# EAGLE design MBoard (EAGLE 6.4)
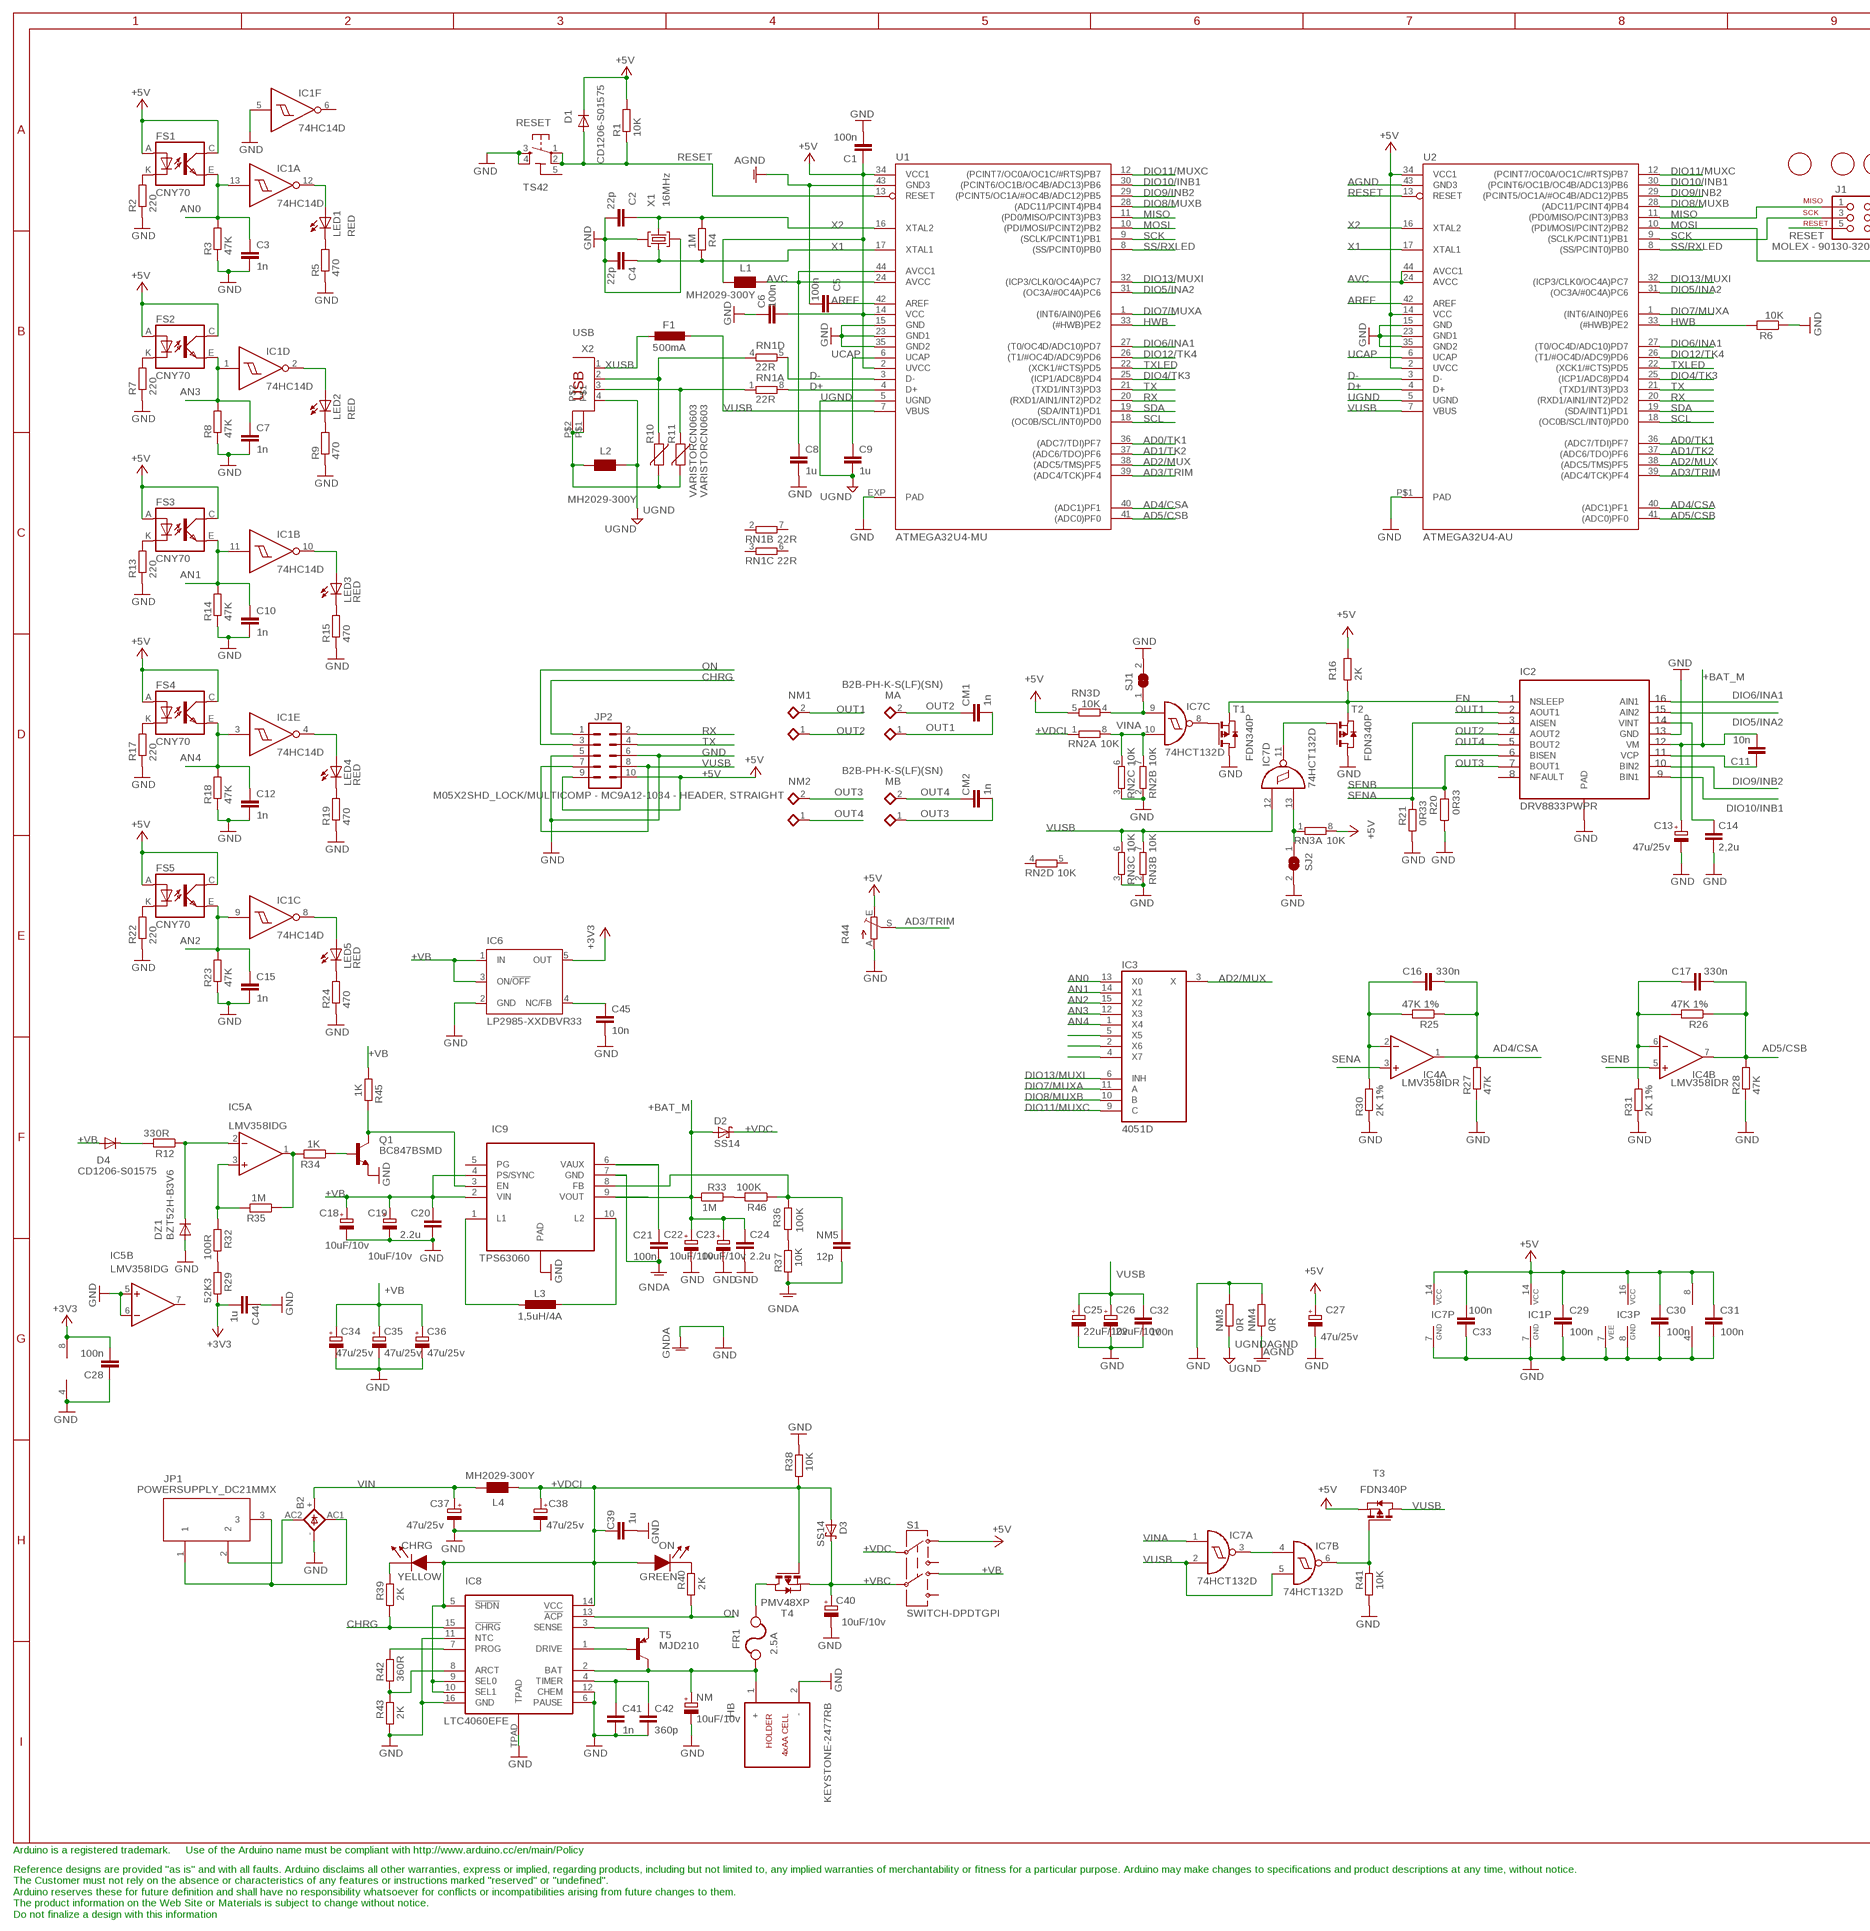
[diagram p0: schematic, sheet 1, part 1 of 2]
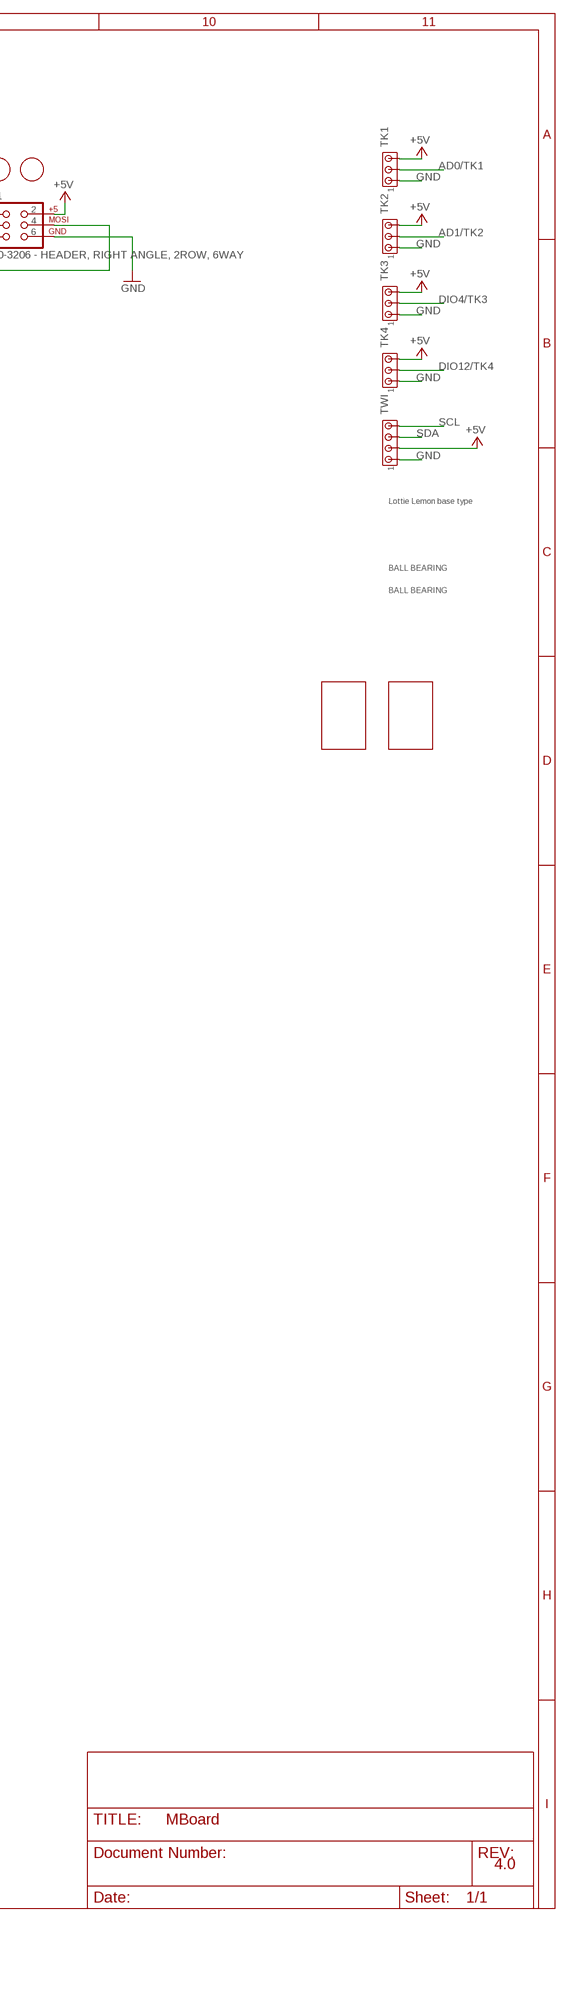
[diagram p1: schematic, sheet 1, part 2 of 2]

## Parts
B2  KBL  [KBL]
BB1  LOTTIE_LEMON_BALL_BEARING  [BALL_BEARING_LOTTIE_LEMON]
BB2  LOTTIE_LEMON_BALL_BEARING  [BALL_BEARING_LOTTIE_LEMON]
C1  100n  C-EUC0603  [C0603-ROUND]
C2  22p  C-EUC0603  [C0603-ROUND]
C3  1n  C-EUC0603  [C0603-ROUND]
C4  22p  C-EUC0603  [C0603-ROUND]
C5  100n  C-EUC0603  [C0603-ROUND]
C6  100n  C-EUC0603  [C0603-ROUND]
C7  1n  C-EUC0603  [C0603-ROUND]
C8  1u  C-EUC0603  [C0603-ROUND]
C9  1u  C-EUC0603  [C0603-ROUND]
C10  1n  C-EUC0603  [C0603-ROUND]
C11  10n  C-EUC0603  [C0603-ROUND]
C12  1n  C-EUC0603  [C0603-ROUND]
C13  47u/25v  CPOL-EUD  [PANASONIC_D]
C14  2,2u  C-EUC0805K  [C0805K]
C15  1n  C-EUC0603  [C0603-ROUND]
C16  330n  C-EUC0603  [C0603-ROUND]
C17  330n  C-EUC0603  [C0603-ROUND]
C18  10uF/10v  CPOL-EUSMCB  [SMC_B]
C19  10uF/10v  CPOL-EUSMCB  [SMC_B]
C20  2.2u  C-EUC0805K  [C0805K]
C21  100n  C-EUC0603  [C0603-ROUND]
C22  10uF/10v  CPOL-EUSMCB  [SMC_B]
C23  10uF/10v  CPOL-EUSMCB  [SMC_B]
C24  2.2u  C-EUC0805K  [C0805K]
C25  22uF/10v  CPOL-EUSMCB  [SMC_B]
C26  22uF/10v  CPOL-EUSMCB  [SMC_B]
C27  47u/25v  CPOL-EUD  [PANASONIC_D]
C28  100n  C-EUC0603  [C0603-ROUND]
C29  100n  C-EUC0603  [C0603-ROUND]
C30  100n  C-EUC0603  [C0603-ROUND]
C31  100n  C-EUC0603  [C0603-ROUND]
C32  100n  C-EUC0603  [C0603-ROUND]
C33  100n  C-EUC0603  [C0603-ROUND]
C34  47u/25v  CPOL-EUD  [PANASONIC_D]
C35  47u/25v  CPOL-EUD  [PANASONIC_D]
C36  47u/25v  CPOL-EUD  [PANASONIC_D]
C37  47u/25v  CPOL-EUD  [PANASONIC_D]
C38  47u/25v  CPOL-EUD  [PANASONIC_D]
C39  1u  C-EUC0603  [C0603-ROUND]
C40  10uF/10v  CPOL-EUSMCB  [SMC_B]
C41  1n  C-EUC0603  [C0603-ROUND]
C42  360p  C-EUC0603  [C0603-ROUND]
C44  1u  C-EUC0603  [C0603-ROUND]
C45  10n  C-EU0603-RND  [C0603-ROUND]
CHRG  YELLOW  MYSMD_LED0805  [SMD_LED0805]
CM1  1n  C-EUC0603  [C0603-ROUND]
CM2  1n  C-EUC0603  [C0603-ROUND]
D1  CD1206-S01575  DIODE-MINIMELF  [MINIMELF]
D2  SS14  SCHOTTKY-DIODESMD  [SMB@1]
D3  SS14  SCHOTTKY-DIODESMD  [SMB@1]
D4  CD1206-S01575  DIODE-MINIMELF  [MINIMELF]
DZ1  BZT52H-B3V6  DIODE-SOD123  [SOD123]
F1  500mA  L-EUL1812  [L1812]
FM1  FIDUCIALMOUNT  [FIDUCIA-MOUNT]
FM2  FIDUCIALMOUNT  [FIDUCIA-MOUNT]
FM3  FIDUCIALMOUNT  [FIDUCIA-MOUNT]
FR1  2.5A  PTC_RESETTABLE_FUSES  [MF-MSMF-S2]
FS1  CNY70  [4]
FS2  CNY70  [4]
FS3  CNY70  [4]
FS4  CNY70  [4]
FS5  CNY70  [4]
HB  KEYSTONE-2477RB  4XAA-BATTERY_HOLDER  [4XAA_BATTERY-HOLDER]
IC1  74HC14D  [SO14]
IC2  DRV8833PWPR  DRV8833  [R-PDSO-G16]
IC3  4051D  [SO16]
IC4  LMV358IDR  LMV358MX  [SO08@1]
IC5  LMV358IDG  LM358D  [SO08]
IC6  LP2985-XXDBVR33  [SOT23-DBV]
IC7  74HCT132D  [SO14]
IC8  LTC4060EFE  LTC4060  [TSSOP16]
IC9  TPS63060  [R-PVSON-10N]
J1  MOLEX - 90130-3206 - HEADER, RIGHT ANGLE, 2ROW, 6WAY  AVR_SPI_PRG_6PTH  [2X3]
JP1  POWERSUPPLY_DC21MMX  [POWERSUPPLY_DC-21MM]
JP2  M05X2SHD_LOCK/MULTICOMP - MC9A12-1034 - HEADER, STRAIGHT  M05X2SHD_LOCK  [2X5-SHROUDED_LOCK]
L1  MH2029-300Y  WE-CBF_0805  [0805]
L2  MH2029-300Y  WE-CBF_0805  [0805]
L3  1,5uH/4A  L-EUWE-TPC  [POWER-CHOKE_WE-TPC]
L4  MH2029-300Y  WE-CBF_0805  [0805]
LED1  RED  LEDCHIP-LED0805  [CHIP-LED0805]
LED2  RED  LEDCHIP-LED0805  [CHIP-LED0805]
LED3  RED  LEDCHIP-LED0805  [CHIP-LED0805]
LED4  RED  LEDCHIP-LED0805  [CHIP-LED0805]
LED5  RED  LEDCHIP-LED0805  [CHIP-LED0805]
LL1  LOTTIE_LEMON_DC_MOTOR_48X_L  [CARCASA_MOTOR_L_LOTTIE_LEMON]
MA  B2B-PH-K-S(LF)(SN)  B2B-PH-KL  [B2B-PH_KL]
MB  B2B-PH-K-S(LF)(SN)  B2B-PH-KL  [B2B-PH_KL]
NM  10uF/10v  CPOL-EUSMCB  [SMC_B]
NM1  B2B-PH-K-S(LF)(SN)  B2B-PH-KL  [B2B-PH_KL]
NM2  B2B-PH-K-S(LF)(SN)  B2B-PH-KL  [B2B-PH_KL]
NM3  0R  R-EU_R0805  [R0805]
NM4  0R  R-EU_R0805  [R0805]
NM5  12p  C-EUC0603  [C0603-ROUND]
ON  GREEN  MYSMD_LED0805  [SMD_LED0805]
Q1  BC847BSMD  [SOT23]
R1  10K  R-EU_0603-RND  [R0603-ROUND]
R2  220  R-EU_R0603  [R0603-ROUND]
R3  47K  R-EU_R0603  [R0603-ROUND]
R4  1M  R-EU_0603-RND  [R0603-ROUND]
R5  470  R-EU_R0603  [R0603-ROUND]
R6  10K  R-EU_0603-RND  [R0603-ROUND]
R7  220  R-EU_R0603  [R0603-ROUND]
R8  47K  R-EU_0603-RND  [R0603-ROUND]
R9  470  R-EU_0603-RND  [R0603-ROUND]
R10  VARISTORCN0603  [CT/CN0603]
R11  VARISTORCN0603  [CT/CN0603]
R12  330R  R-EU_0603-RND  [R0603-ROUND]
R13  220  R-EU_R0603  [R0603-ROUND]
R14  47K  R-EU_R0603  [R0603-ROUND]
R15  470  R-EU_R0603  [R0603-ROUND]
R16  2K  R-EU_0603-RND  [R0603-ROUND]
R17  220  R-EU_R0603  [R0603-ROUND]
R18  47K  R-EU_R0603  [R0603-ROUND]
R19  470  R-EU_R0603  [R0603-ROUND]
R20  0R33  R-EU_R1206  [R1206]
R21  0R33  R-EU_R1206  [R1206]
R22  220  R-EU_R0603  [R0603-ROUND]
R23  47K  R-EU_R0603  [R0603-ROUND]
R24  470  R-EU_R0603  [R0603-ROUND]
R25  47K 1%  R-EU_0603-RND  [R0603-ROUND]
R26  47K 1%  R-EU_0603-RND  [R0603-ROUND]
R27  47K  R-EU_0603-RND  [R0603-ROUND]
R28  47K  R-EU_0603-RND  [R0603-ROUND]
R29  52K3  R-EU_0603-RND  [R0603-ROUND]
R30  2K 1%  R-EU_0603-RND  [R0603-ROUND]
R31  2K 1%  R-EU_0603-RND  [R0603-ROUND]
R32  100R  R-EU_0603-RND  [R0603-ROUND]
R33  1M  R-EU_0603-RND  [R0603-ROUND]
R34  1K  R-EU_0603-RND  [R0603-ROUND]
R35  1M  R-EU_0603-RND  [R0603-ROUND]
R36  100K  R-EU_0603-RND  [R0603-ROUND]
R37  10K  R-EU_0603-RND  [R0603-ROUND]
R38  10K  R-EU_0603-RND  [R0603-ROUND]
R39  2K  R-EU_0603-RND  [R0603-ROUND]
R40  2K  R-EU_0603-RND  [R0603-ROUND]
R41  10K  R-EU_0603-RND  [R0603-ROUND]
R42  360R  R-EU_0603-RND  [R0603-ROUND]
R43  2K  R-EU_0603-RND  [R0603-ROUND]
R44  TRIM_EU-CA9V  [CA9V]
R45  1K  R-EU_0603-RND  [R0603-ROUND]
R46  100K  R-EU_0603-RND  [R0603-ROUND]
RESET  TS42  [TS42]
RN1  22R  4R-NCAY16  [CAY16]
RN2  10K  4R-NCAY16  [CAY16]
RN3  10K  4R-NCAY16  [CAY16]
RR1  LOTTIE_LEMON_DC_MOTOR_48X_R  [CARCASA_MOTOR_R_LOTTIE_LEMON]
S1  SWITCH-DPDTGPI  [GPI-152-3013]
SJ1  SJL  [SJL]
SJ2  SJL  [SJL]
T1  FDN340P  PMOSSOT23  [SOT-23]
T2  FDN340P  PMOSSOT23  [SOT-23]
T3  FDN340P  PMOSSOT23  [SOT-23]
T4  PMV48XP  PMOSSOT23  [SOT-23]
T5  MJD210  MJD32  [DPAK]
TK1  MTA03-100  [10X03MTA]
TK2  MTA03-100  [10X03MTA]
TK3  MTA03-100  [10X03MTA]
TK4  MTA03-100  [10X03MTA]
TWI  MTA04-100  [10X04MTA]
U1  ATMEGA32U4-MU  ATMEGA32U4-XUMU  [QFN44ML7X7]
U2  ATMEGA32U4-AU  ATMEGA32U4-XUAU  [TQFP44-PAD]
U$1  LOTTIE_LEMON_BASE_TYPE  [BASE_ROBOT_001]
U$2  LOTTIE_LEMON_PADS  [PADS_LOTTIE_LEMON]
W1  LOTTIE_LEMON_WHEEL  [WHEEL_LOTTIE_LEMON]
W2  LOTTIE_LEMON_WHEEL  [WHEEL_LOTTIE_LEMON]
X1  16MHz  CRYSTAL-3.2-2.5  [CRYSTAL-3.2-2.5]
X2  USB  PN61729  [PN61729]

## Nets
+3V3: C28.2 C44.1 IC5.8(P:V+) IC6.5(OUT) R29.2
+5V [+5v]: C1.1 C6.2 C27.+ C29.1 C30.1 C31.1 C33.2 D1.C FS1.A FS1.C(COL) FS2.A FS2.C(COL) FS3.A FS3.C(COL) FS4.A FS4.C(COL) FS5.A FS5.C(COL) IC1.14(P:VCC) IC3.16(VCC) IC4.8(P:V+) IC7.14(P:VCC) J1.2 JP2.9 JP2.10 L1.1 R1.2 R16.2 R44.E RN3.5 RN3.8 S1.10 T3.2(S) TK1.3 TK2.3 TK3.3 TK4.3 TWI.2 U1.2(UVCC) U1.14(VCC) U1.34(VCC1) U2.2(UVCC) U2.14(VCC) U2.34(VCC1)
+BAT_M [power]: C11.2 C13.+ C22.+ C23.+ C24.1 D2.A IC2.P$12(VM) IC9.9(VOUT) R33.1
+VB [power]: C18.+ C19.+ C20.1 C34.+ C35.+ C36.+ D4.A IC6.1(IN) IC6.3(ON/!OFF) IC9.2(VIN) IC9.4(PS/SYNC) R45.1 S1.11
+VBC [+5v]: C40.+ D3.C S1.C@2 T4.2(S)
+VDC [+5v]: D2.C S1.C@1
+VDCI [power]: C38.+ C39.2 CHRG.2(AN) D3.A IC8.5(!SHDN) IC8.9(SEL0) IC8.10(SEL1) IC8.14(VCC) L4.2 ON.2(AN) R38.1 RN2.1 T4.3(G)
AD0/TK1: TK1.2 U1.36((ADC7/TDI)PF7) U2.36((ADC7/TDI)PF7)
AD1/TK2: TK2.2 U1.37((ADC6/TDO)PF6) U2.37((ADC6/TDO)PF6)
AD2/MUX: IC3.3(X) U1.38((ADC5/TMS)PF5) U2.38((ADC5/TMS)PF5)
AD3/TRIM: R44.S U1.39((ADC4/TCK)PF4) U2.39((ADC4/TCK)PF4)
AD4/CSA: C16.2 IC4.1(A:OUT) R25.1 R27.2 U1.40((ADC1)PF1) U2.40((ADC1)PF1)
AD5/CSB: C17.2 IC4.7(B:OUT) R26.1 R28.2 U1.41((ADC0)PF0) U2.41((ADC0)PF0)
AGND: C5.2 NM4.1 U1.43(GND3) U2.43(GND3)
AN0: C3.1 FS1.E(EMI) IC1.13(A:I) IC3.13(X0) R3.2
AN1: C10.1 FS3.E(EMI) IC1.11(B:I) IC3.14(X1) R14.2
AN2: C15.1 FS5.E(EMI) IC1.9(C:I) IC3.15(X2) R23.2
AN3: C7.1 FS2.E(EMI) IC1.1(D:I) IC3.12(X3) R8.2
AN4: C12.1 FS4.E(EMI) IC1.3(E:I) IC3.1(X4) R18.2
AREF: C5.1 U1.42(AREF) U2.42(AREF)
AVC: C8.1 L1.2 U1.24(AVCC) U1.44(AVCC1) U2.24(AVCC) U2.44(AVCC1)
CHRG: IC8.15(!CHRG) JP2.1 R39.1
D+: RN1.8 U1.4(D+) U2.4(D+)
D-: RN1.5 U1.3(D-) U2.3(D-)
DIO4/TK3: TK3.2 U1.25((ICP1/ADC8)PD4) U2.25((ICP1/ADC8)PD4)
DIO5/INA2: IC2.P$15(AIN2) U1.31((OC3A/#0C4A)PC6) U2.31((OC3A/#0C4A)PC6)
DIO6/INA1: IC2.P$16(AIN1) U1.27((T0/OC4D/ADC10)PD7) U2.27((T0/OC4D/ADC10)PD7)
DIO7/MUXA: IC3.11(A) U1.1((INT6/AIN0)PE6) U2.1((INT6/AIN0)PE6)
DIO8/MUXB: IC3.10(B) U1.28((ADC11/PCINT4)PB4) U2.28((ADC11/PCINT4)PB4)
DIO9/INB2: IC2.P$10(BIN2) U1.29((PCINT5/OC1A/#OC4B/ADC12)PB5) U2.29((PCINT5/OC1A/#OC4B/ADC12)PB5)
DIO10/INB1: IC2.P$9(BIN1) U1.30((PCINT6/OC1B/OC4B/ADC13)PB6) U2.30((PCINT6/OC1B/OC4B/ADC13)PB6)
DIO11/MUXC: IC3.9(C) U1.12((PCINT7/OC0A/OC1C/#RTS)PB7) U2.12((PCINT7/OC0A/OC1C/#RTS)PB7)
DIO12/TK4: TK4.2 U1.26((T1/#OC4D/ADC9)PD6) U2.26((T1/#OC4D/ADC9)PD6)
DIO13/MUXI: IC3.6(INH) U1.32((ICP3/CLK0/OC4A)PC7) U2.32((ICP3/CLK0/OC4A)PC7)
EN [+5v]: IC2.P$1(NSLEEP) R16.1 T1.2(S) T2.2(S)
GND [gnd]: B2.- C1.2 C2.2 C3.2 C4.2 C6.1 C7.2 C8.2 C10.2 C12.2 C13.- C14.2 C15.2 C18.- C19.- C20.2 C22.- C23.- C24.2 C25.- C26.- C27.- C28.1 C29.2 C30.2 C31.2 C32.1 C33.1 C34.- C35.- C36.- C37.- C38.- C39.1 C40.- C41.2 C42.2 C44.2 C45.2 DZ1.A HB.2(-) IC1.5(F:I) IC1.7(P:GND) IC2.P$13(GND) IC2.P$17(PAD) IC3.7(VEE) IC3.8(GND) IC4.4(P:V-) IC5.4(P:V-) IC5.5(B:+IN) IC5.6(B:-IN) IC6.2(GND) IC7.7(P:GND) IC8.6(PAUSE) IC8.11(NTC) IC8.12(CHEM) IC8.16(GND) IC8.TPAD IC9.PAD J1.6 JP2.5 JP2.6 NM3.2 NM4.2 NM.- Q1.2(E) R2.1 R3.1 R5.1 R6.1 R7.1 R8.1 R9.1 R13.1 R14.1 R15.1 R17.1 R18.1 R19.1 R20.1 R21.1 R22.1 R23.1 R24.1 R27.1 R28.1 R30.1 R31.1 R38.2 R41.1 R43.1 R44.A RESET.3 RESET.4 RN2.2 RN2.3 RN3.2 RN3.3 SJ1.2 SJ2.2 T1.1(D) T2.1(D) TK1.1 TK2.1 TK3.1 TK4.1 TWI.1 U1.15(GND) U1.23(GND1) U1.35(GND2) U1.EXP(PAD) U2.15(GND) U2.23(GND1) U2.35(GND2) U2.P$1(PAD) X1.2(GND) X1.4(GND)
GNDA [gnd]: C21.2 IC9.7(GND) NM5.2 R37.1 ; supply symbol labelled GND
HWB: R6.2 U1.33((#HWB)PE2) U2.33((#HWB)PE2)
MISO: J1.1 U1.11((PD0/MISO/PCINT3)PB3) U2.11((PD0/MISO/PCINT3)PB3)
MOSI: J1.4 U1.10((PDI/MOSI/PCINT2)PB2) U2.10((PDI/MOSI/PCINT2)PB2)
N$1: CHRG.1(CA) R39.2
N$2: IC3.5(X5)
N$3: IC7.3(A:O) IC7.4(B:I0)
N$4 [power]: B2.AC2(AC1) JP1.2
N$5: IC1.12(A:O) LED1.A
N$6: IC1.10(B:O) LED3.A
N$7 [power]: B2.AC1(AC2) JP1.1 JP1.3
N$8: IC3.2(X6)
N$9: L2.1 R10.2 R11.2 X2.P$1 X2.P$2
N$10: IC3.4(X7)
N$11: IC7.13(D:I1) RN3.1 SJ2.1
N$12: IC9.10(L2) L3.2
N$13: IC8.8(ARCT) R42.1 R43.2
N$14: FS1.K(C) R2.2
N$15: FS3.K(C) R13.2
N$16: LED1.C R5.2
N$17: IC8.7(PROG) R42.2
N$18: LED3.C R15.2
N$19: FS5.K(C) R22.2
N$20: FS2.K(C) R7.2
N$21: IC7.6(B:O) R41.2 T3.3(G)
N$22: LED5.C R24.2
N$23: C11.1 IC2.P$11(VCP)
N$24: FS4.K(C) R17.2
N$25: LED4.C R19.2
N$26: LED2.C R9.2
N$27: IC8.3(SENSE) T5.3(E)
N$28: C17.1 IC4.6(B:-IN) R26.2 R31.2
N$29: C16.1 IC4.2(A:-IN) R25.2 R30.2
N$30: IC7.8(C:O) T1.3(G)
N$31: IC8.1(DRIVE) T5.1(B)
N$32: ON.1(CA) R40.2
N$33: FR1.P$1 HB.1(+) IC8.2(BAT) NM.+ T5.4(C)
N$34: C41.1 C42.1 IC8.4(TIMER)
N$35: C21.1 IC9.6(VAUX)
N$36: IC1.8(C:O) LED5.A
N$37: IC1.2(D:O) LED2.A
N$38: IC1.4(E:O) LED4.A
N$39: IC9.8(FB) NM5.1 R36.1 R46.1
N$40: IC7.11(D:O) T2.3(G)
N$41: C45.1 IC6.4(NC/FB)
N$42: C14.1 IC2.P$14(VINT)
N$43: R36.2 R37.2
N$44: IC7.9(C:I0) RN3.4 SJ1.1
N$45: IC5.3(A:+IN) R32.1 R35.2
N$46: FR1.P$2 T4.1(D)
N$47: IC9.1(L1) L3.1
N$48: DZ1.C IC5.2(A:-IN) R12.1
N$49: R29.1 R32.2
N$50: IC9.3(EN) Q1.3(C) R45.2
N$51: R11.1 RN1.1 X2.3
N$52: IC5.1(A:OUT) R34.2 R35.1
N$53: Q1.1(B) R34.1
N$54: R10.1 RN1.4 X2.2
N$55: D4.C R12.2
N$56: R33.2 R46.2
ON: IC8.13(!ACP) JP2.3 R40.1
OUT1: CM1.2 IC2.P$2(AOUT1) MA.1 NM1.2
OUT2: CM1.1 IC2.P$4(AOUT2) MA.2 NM1.1
OUT3: CM2.1 IC2.P$7(BOUT1) MB.1 NM2.2
OUT4: CM2.2 IC2.P$5(BOUT2) MB.2 NM2.1
RESET: D1.A J1.5 R1.1 RESET.1 RESET.2 U1.13(RESET) U2.13(RESET)
RX: JP2.2 U1.20((RXD1/AIN1/INT2)PD2) U2.20((RXD1/AIN1/INT2)PD2)
SCK: J1.3 U1.9((SCLK/PCINT1)PB1) U2.9((SCLK/PCINT1)PB1)
SCL: TWI.4 U1.18((OC0B/SCL/INT0)PD0) U2.18((OC0B/SCL/INT0)PD0)
SDA: TWI.3 U1.19((SDA/INT1)PD1) U2.19((SDA/INT1)PD1)
SENA: IC2.P$3(AISEN) IC4.3(A:+IN) R21.2
SENB: IC2.P$6(BISEN) IC4.5(B:+IN) R20.2
SS/RXLED: U1.8((SS/PCINT0)PB0) U2.8((SS/PCINT0)PB0)
TX: JP2.4 U1.21((TXD1/INT3)PD3) U2.21((TXD1/INT3)PD3)
TXLED: U1.22((XCK1/#CTS)PD5) U2.22((XCK1/#CTS)PD5)
UCAP: C9.1 U1.6(UCAP) U2.6(UCAP)
UGND: C9.2 L2.2 NM3.1 U1.5(UGND) U2.5(UGND) X2.4
VIN: B2.+ C37.+ L4.1
VINA: IC7.1(A:I0) IC7.10(C:I1) RN2.6 RN2.7 RN2.8
VUSB [usbvcc]: C25.+ C26.+ C32.2 F1.2 IC7.2(A:I1) IC7.5(B:I1) IC7.12(D:I0) JP2.7 JP2.8 RN3.6 RN3.7 T3.1(D) U1.7(VBUS) U2.7(VBUS)
X1: C4.1 R4.2 U1.17(XTAL1) U2.17(XTAL1) X1.1(C1)
X2: C2.1 R4.1 U1.16(XTAL2) U2.16(XTAL2) X1.3(C2)
XUSB: F1.1 X2.1
Unconnected: IC1.6(F:O) IC2.P$8(NFAULT) IC5.7(B:OUT) IC9.5(PG) RN1.2 RN1.3 RN1.6 RN1.7 RN2.4 RN2.5 S1.20 S1.21

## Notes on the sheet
- 4.0
- Arduino is a registered trademark. | Use of the Arduino name must be compliant with http://www.arduino.cc/en/main/Policy
- Reference designs are provided "as is" and with all faults. Arduino disclaims all other warranties, express or implied, regarding products, including but not limited to, any implied warranties of merchantability or fitness for a particular purpose. Arduino may make changes to specifications and product descriptions at any time, without notice. 
  The Customer must not rely on the absence or characteristics of any features or instructions marked "reserved" or "undefined". 
  Arduino reserves these for future definition and shall have no responsibility whatsoever for conflicts or incompatibilities arising from future changes to them. 
  The product information on the Web Site or Materials is subject to change without notice. 
  Do not finalize a design with this information

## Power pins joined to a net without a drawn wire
5-GND: RESET.5(5-GND)

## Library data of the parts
B2 = Smartprj:KBL: DIOTEC RECTIFIER
BB1 BB2 = complubot:LOTTIE_LEMON_BALL_BEARING: BALL WHEEL FOR ROBOT
C1-C12 C14-C17 C20 C21 C24 C28-C33 C39 C41 C42 C44 C45 CM1 CM2 NM5 = Smartprj:C-EU: CAPACITOR, European symbol
C13 C18 C19 C22 C23 C25-C27 C34-C38 C40 NM = Smartprj:CPOL-EU: POLARIZED CAPACITOR, European symbol
CHRG ON = Smartprj:MYSMD_LED0805
D1 D4 DZ1 = diode:DIODE-: DIODE
D2 D3 = diode:SCHOTTKY-DIODE: Schottky Diode
F1 = rcl:L-EU: INDUCTOR, European symbol
FM1-FM3 = Smartprj:FIDUCIALMOUNT
FR1 = Smartprj:PTC_RESETTABLE_FUSES
FS1-FS5 = cny70:CNY70
HB = Smartprj:4XAA-BATTERY_HOLDER: KEYSTONE 4xAA Battery Holder
IC1 = 74xx-eu:74*14: Hex schmitt trigger INVERTER
IC2 = Smartprj:DRV8833: DRV883 Dual H DC/STEPPER Motor Drive Ti
IC3 = 40xx:4051: 8-channel ANALOG MULTIPLEXER
IC4 = linear:LMV358?*: Dual General Purpose, Low Voltage, Rail-to-Rail Output Operational Amplifiers Source: http://www.national.com/mpf/LM/LMV321.html http://www.national.com/dt/lmv_qual.pdf
IC5 = Smartprj:LM358: OP AMP also LM158; LM258; LM2904 Source: http://cache.national.com/ds/LM/LM158.pdf
IC6 = Smartprj:LP2985-XXDBVR: ULTRALOW-POWER 50-mA LOW-DROPOUT LINEAR REGULATORS 50-mA Low-Dropout Regulator Source: http://focus.ti.com/lit/ds/symlink/tps77001.pdf
IC7 = 74xx-eu:74*132: Quad 2-input NAND schmitt trigger
IC8 = Smartprj:LTC4060: LTC4060 Standalone Linear NiMH/NiCd 1 to 4 cells Fast Battery Charger LINEAR-TECHNOLOGY (LT)
IC9 = Smartprj:TPS63060: TPS63060 Single Inductor Buck-Boost Converter 2A Switches
J1 = SparkFun:AVR_SPI_PRG_6: AVR ISP 6 Pin This is the reduced ISP connector for AVR programming. Common on Arduino. This footprint will take up less PCB space and can be used with a 10-pin to 6-pin adapter such as SKU: BOB-08508
JP1 = Smartprj:POWERSUPPLY_DC21MM
JP2 = Smartprj:M05X2: Header 5x2 Standard 10-pin dual row 0.1" header. Commonly used with AVR-ISP. Use with Spark Fun Electronics SKU: PRT-00778
L1 L2 L4 = wuerth-elektronik:WE-CBF: SMD EMI Suppression Ferrite Beads
L3 = Smartprj:L-EU: INDUCTOR, European symbol
LED1-LED5 = led:LED: LED
LL1 = complubot1:LOTTIE_LEMON_DC_MOTOR_48X_L: MOTOR DC GEAR 48X L
MA MB NM1 NM2 = Smartprj:B2B-PH-KL: PH Connectors Two Wire Connector
NM3 NM4 = resistor:R-EU_: RESISTOR, European symbol
Q1 = transistor-npn:BC847*: NPN Transistor
R1-R9 R12-R43 R45 R46 = Smartprj:R-EU_: RESISTOR, European symbol
R10 R11 = varistor:VARISTOR: VARISTOR
R44 = pot:TRIM_EU-: POTENTIOMETER
RESET = Smartprj:TS42: TS42 Dongnan Electronics Tact switch VDC 12V - 50mA
RN1-RN3 = resistor-dil:4R-N: Array Chip Resistor Source: RS Component / Phycomp
RR1 = complubot1:LOTTIE_LEMON_DC_MOTOR_48X_R: MOTOR DC GEAR 48X R
S1 = SparkFun:SWITCH-DPDT: DPDT Version of the COM-00597
SJ1 SJ2 = Smartprj:SJ: SMD solder JUMPER
T1-T4 = Smartprj:PMOSSOT23: MOS FET
T5 = transistor:MJD32*: Complementary Power Transistors
TK1-TK4 = con-amp:MTA03-100: AMP connector
TWI = con-amp:MTA04-100: AMP connector
U1 U2 = Smartprj:ATMEGA32U4-XU
U$1 = complubot:LOTTIE_LEMON_BASE_TYPE: Lottie Lemon Robot Base
U$2 = complubot:LOTTIE_LEMON_PADS: PADS FOR LOTTIE LEMON
W1 W2 = complubot:LOTTIE_LEMON_WHEEL: WHEEL LOTTIE LEMON
X1 = Smartprj:CRYSTAL-3.2-2.5
X2 = Smartprj:PN61729: BERG USB connector

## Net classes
0 default: width 0.254 mm, drill 0.584 mm, clearance 0.203 mm
1 power: width 0.254 mm, drill 0.584 mm, clearance 0.203 mm
2 gnd: width 0.254 mm, drill 0.584 mm, clearance 0.203 mm
3 usbvcc: width 0.254 mm, drill 0.584 mm, clearance 0.203 mm
5 +5v: width 0.254 mm, drill 0.584 mm, clearance 0.203 mm

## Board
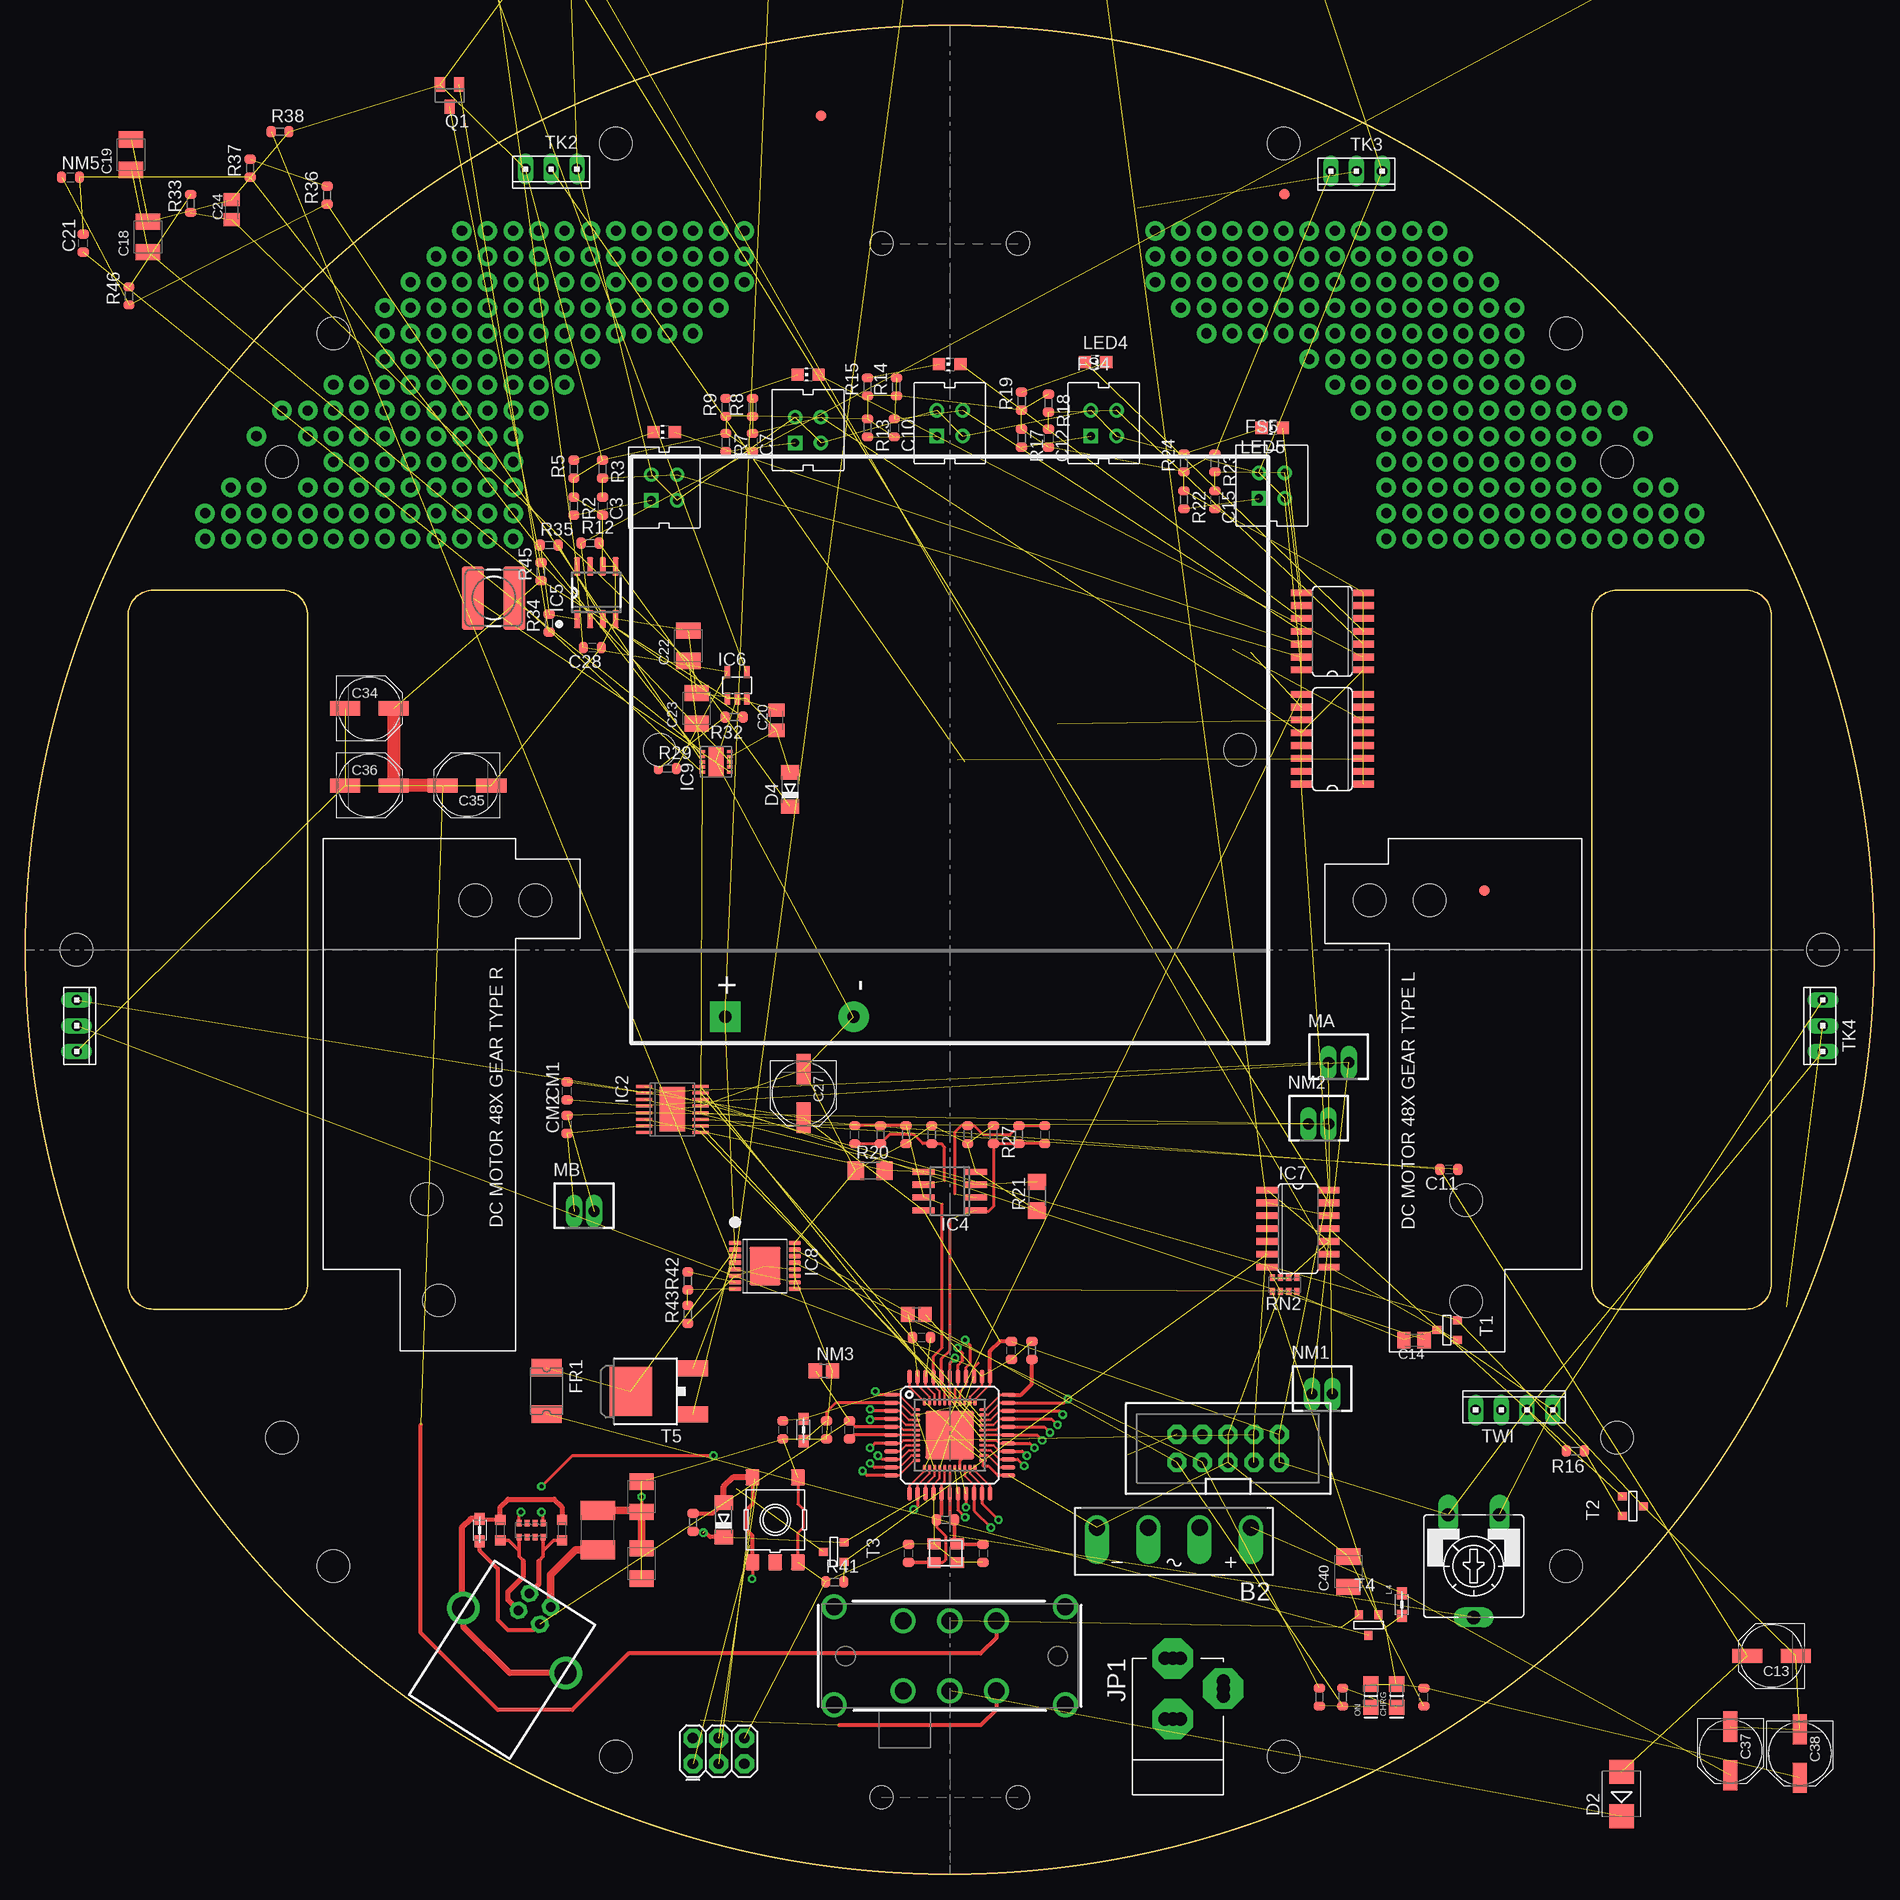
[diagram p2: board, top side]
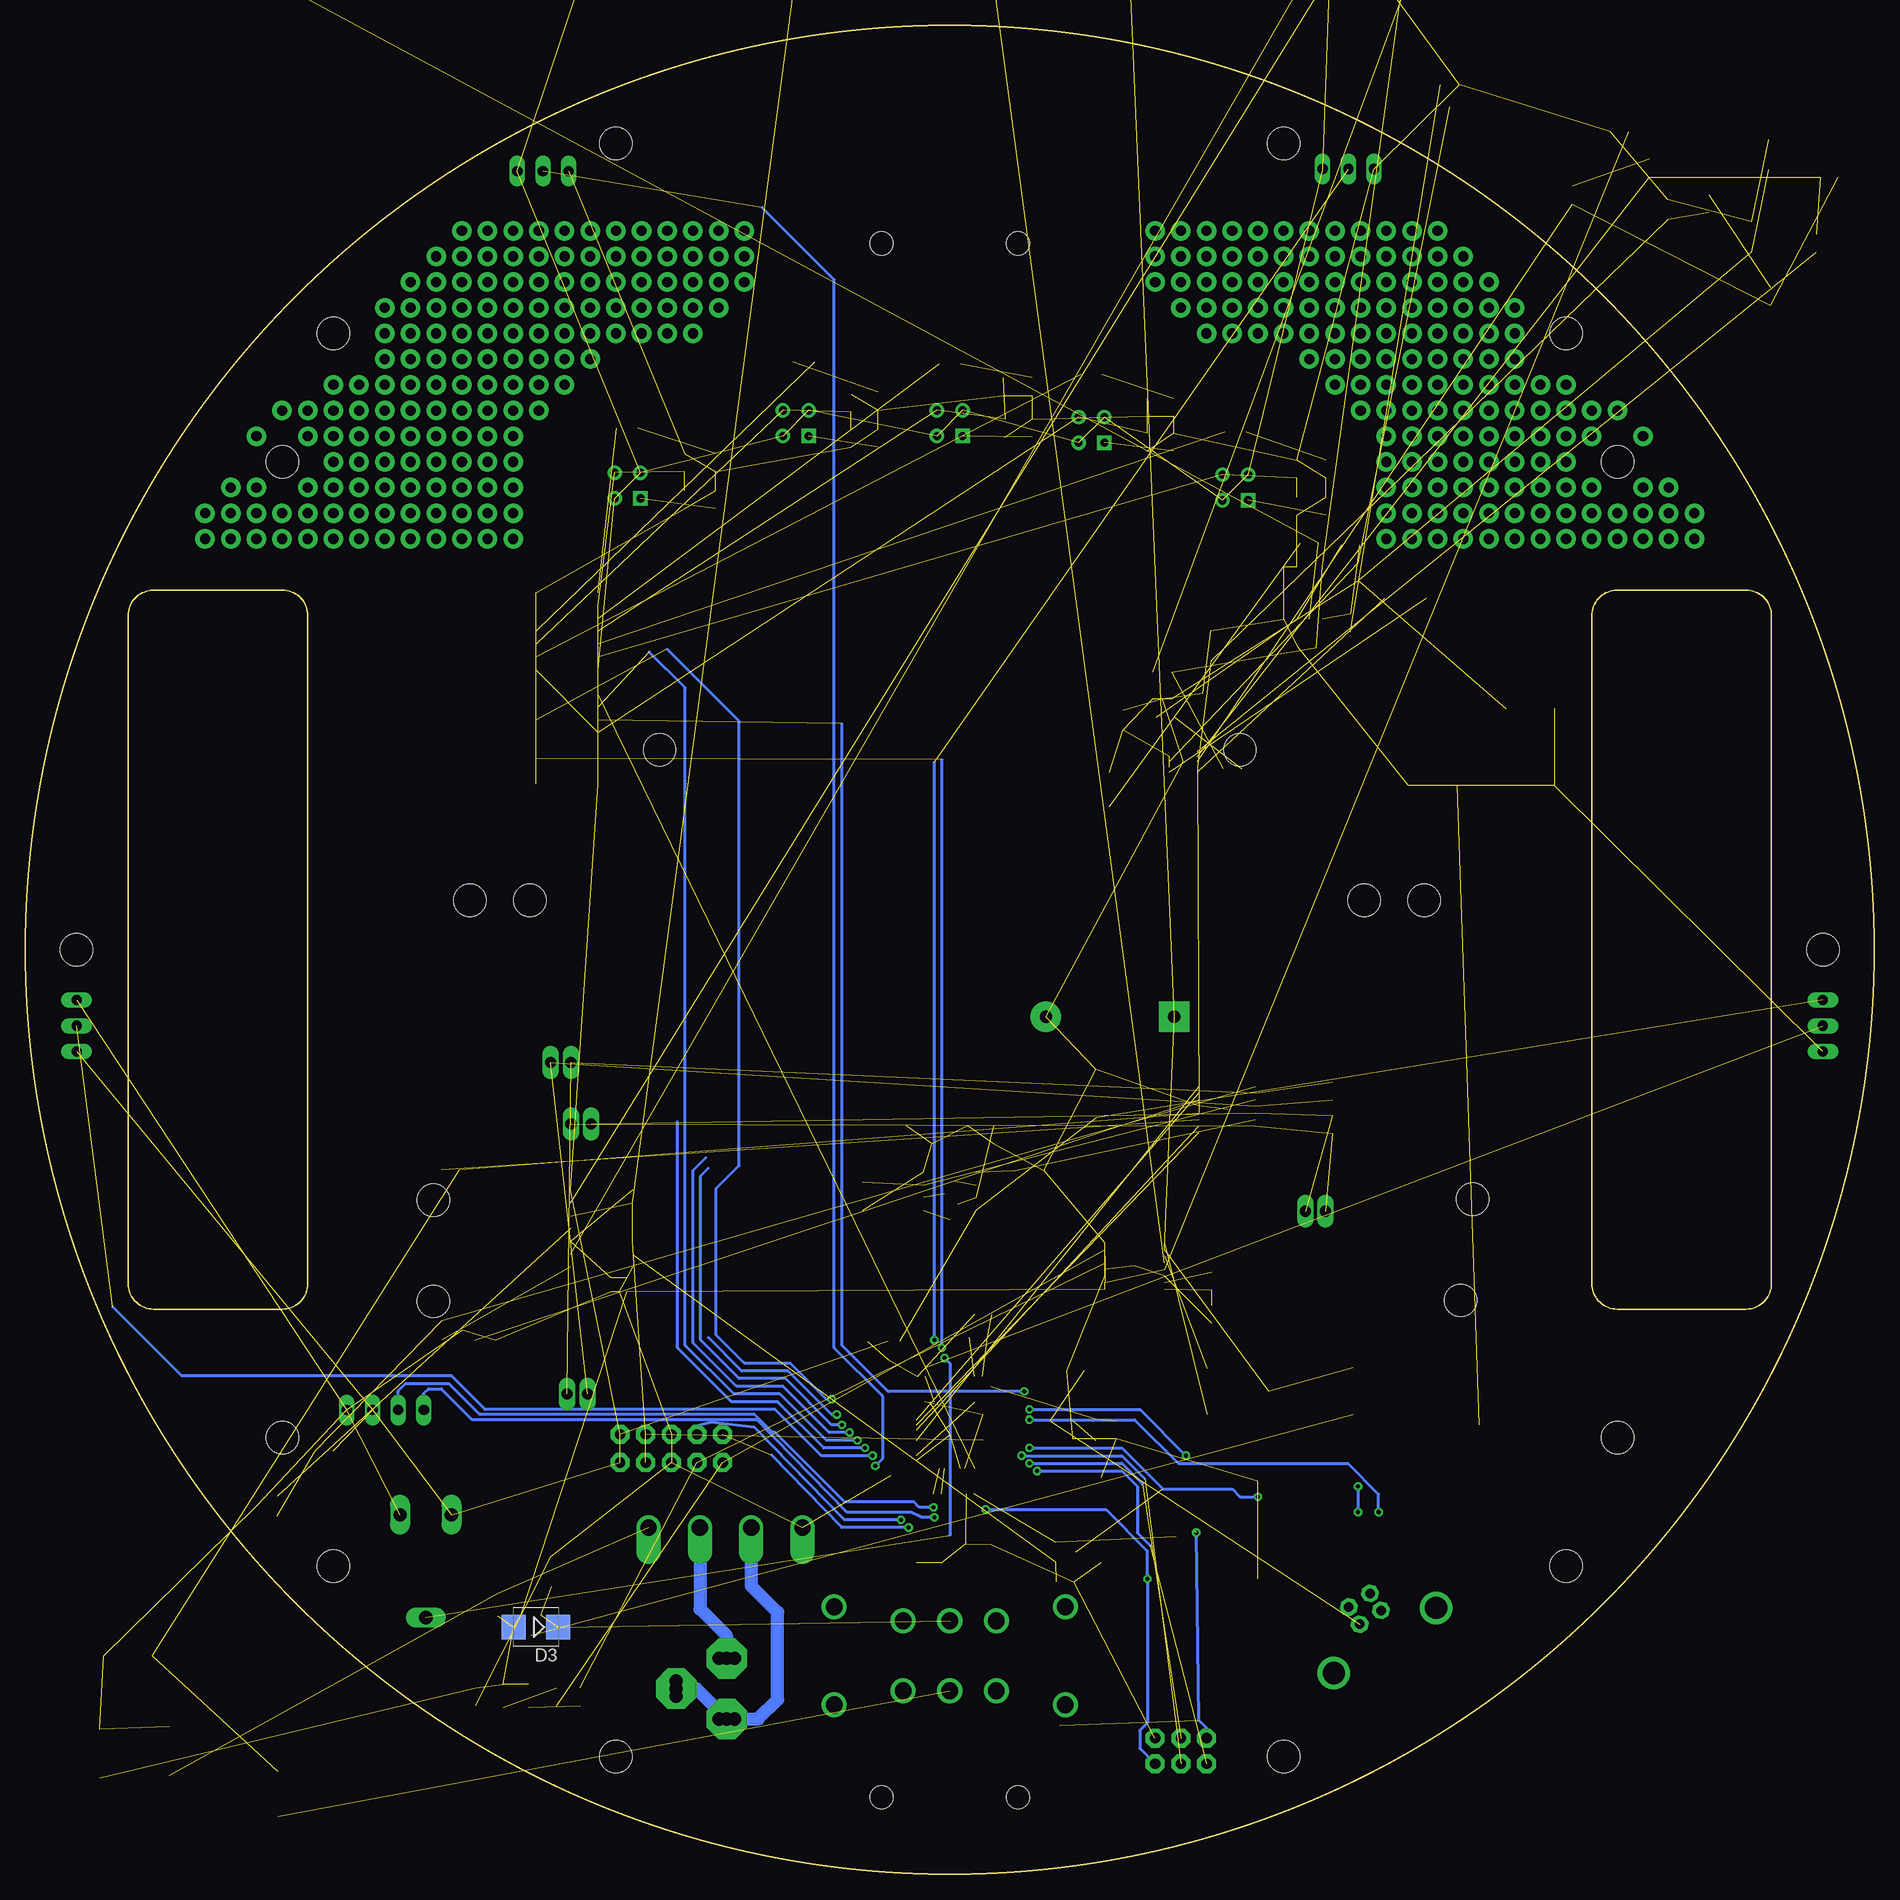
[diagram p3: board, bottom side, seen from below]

Size 182.88 x 182.88 mm. Coordinates in mm from the lower left corner, seen from the top.
Copper layers (1*16): Top 0.035mm / dielectric 1.5mm / Bottom 0.035mm
Design rules "default *": minimum track width 10mil, minimum drill 24mil, track to track 8mil, track to pad 8mil, pad to pad 8mil, via to via 8mil, smd to smd 8mil, copper to edge 30mil, drill to drill 8mil, minimum pad ring 10mil, minimum via ring 8mil, stop-mask expansion 4mil, vias tented up to drill 0mil, thermal gap 10mil

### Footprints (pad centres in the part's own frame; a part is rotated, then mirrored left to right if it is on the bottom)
KBL = drill 1.6 offset: + -7.62,-1.27; - 7.62,-1.27; AC1 2.54,-1.27; AC2 -2.54,-1.27
BALL_BEARING_LOTTIE_LEMON = hole 2.286: -6.731,0; 6.731,0
C0603-ROUND = smd 0.898 x 1.1: 1 -0.889,0; 2 0.889,0
PANASONIC_D = smd 3 x 1.4: + 2.4,0; - -2.4,0
C0805K = smd 1.3 x 1.6: 1 -1,0; 2 1,0
SMC_B = smd 1.6 x 2.4: + -1.5,0; - 1.5,0
SMD_LED0805 = smd 1.524 x 1.524: 1 0,0; 2 2.286,0
MINIMELF = smd 1.4 x 1.8: A 1.7,0; C -1.7,0
SMB@1 = smd 2.4 x 2.4: A 2.2,0; C -2.2,0
SOD123 = smd 1.4 x 1.4: A 1.9,0; C -1.9,0
L1812 = smd 1.9 x 3.4: 1 -1.95,0; 2 1.95,0
FIDUCIA-MOUNT = smd 1.016 x 1.016: P$1 0,0
MF-MSMF-S2 = smd 1.7 x 3: P$1 -2.3,0; P$2 2.3,0
4 = drill 0.8 pad 1.422: A -1.27,1.27; C 1.27,-1.27; E 1.27,1.27 | drill 0.8 pad 1.422 square: K -1.27,-1.27
4XAA_BATTERY-HOLDER = drill 1.2 pad 3 square: 1 26.4,-22.2 | drill 1.2 pad 3: 2 26.4,-9.5 | hole 3.2: 0,28.7; 0,-28.7
SO14 = smd 0.66 x 2.032: 1 -3.81,-3.073; 2 -2.54,-3.073; 3 -1.27,-3.073; 4 0,-3.073; 5 1.27,-3.073; 6 2.54,-3.073; 7 3.81,-3.073; 8 3.81,3.073; 9 2.54,3.073; 10 1.27,3.073; 11 0,3.073; 12 -1.27,3.073; 13 -2.54,3.073; 14 -3.81,3.073
R-PDSO-G16 = smd 0.3 x 1.6: P$1 -2.275,-2.8; P$2 -1.625,-2.8; P$3 -0.975,-2.8; P$4 -0.325,-2.8; P$5 0.325,-2.8; P$6 0.975,-2.8; P$7 1.625,-2.8; P$8 2.275,-2.8; P$9 2.275,2.8; P$10 1.625,2.8; P$11 0.975,2.8; P$12 0.325,2.8; P$13 -0.325,2.8; P$14 -0.975,2.8; P$15 -1.625,2.8; P$16 -2.275,2.8 | smd 4.4 x 2.5: P$17 0,0
SO16 = smd 0.66 x 2.032: 1 -4.445,-3.073; 2 -3.175,-3.073; 3 -1.905,-3.073; 4 -0.635,-3.073; 5 0.635,-3.073; 6 1.905,-3.073; 7 3.175,-3.073; 8 4.445,-3.073; 9 4.445,3.073; 10 3.175,3.073; 11 1.905,3.073; 12 0.635,3.073; 13 -0.635,3.073; 14 -1.905,3.073; 15 -3.175,3.073; 16 -4.445,3.073
SO08@1 = smd 0.6 x 2.2: 1 -1.905,-2.6; 2 -0.635,-2.6; 3 0.635,-2.6; 4 1.905,-2.6; 5 1.905,2.6; 6 0.635,2.6; 7 -0.635,2.6; 8 -1.905,2.6
SO08 = smd 0.6 x 1.8: 1 -1.905,-2.6; 2 -0.635,-2.6; 3 0.635,-2.6; 4 1.905,-2.6; 5 1.905,2.6; 6 0.635,2.6; 7 -0.635,2.6; 8 -1.905,2.6
SOT23-DBV = smd 0.55 x 1.2: 1 -0.95,-1.3; 2 0,-1.3; 3 0.95,-1.3; 4 0.95,1.3; 5 -0.95,1.3
TSSOP16 = smd 0.45 x 1.2: 1 -2.275,-2.95; 2 -1.625,-2.95; 3 -0.975,-2.95; 4 -0.325,-2.95; 5 0.325,-2.95; 6 0.975,-2.95; 7 1.625,-2.95; 8 2.275,-2.95; 9 2.275,2.95; 10 1.625,2.95; 11 0.975,2.95; 12 0.325,2.95; 13 -0.325,2.95; 14 -0.975,2.95; 15 -1.625,2.95; 16 -2.275,2.95 | smd 3.8 x 3.1: TPAD 0,0
R-PVSON-10N = smd 0.3 x 0.65: 1 -1,-1.375; 2 -0.5,-1.375; 3 0,-1.375; 4 0.5,-1.375; 5 1,-1.375; 6 1,1.375; 7 0.5,1.375; 8 0,1.375; 9 -0.5,1.375; 10 -1,1.375 | smd 3 x 1.6: PAD 0,0
2X3 = drill 1.016 pad 1.88 octagon: 1 0,0; 2 0,2.54; 3 2.54,0; 4 2.54,2.54; 5 5.08,0; 6 5.08,2.54
POWERSUPPLY_DC-21MM = drill 1.3 pad 4 octagon: 1 -5.08,-3.353; 2 -0.076,-6.35; 3 -0.076,-0.356 | drill 1.3: 4 -5.08,-4.115; 5 -5.08,-2.591; 6 -0.838,-0.356; 7 0.686,-0.356; 8 -0.838,-6.35; 9 0.686,-6.35
2X5-SHROUDED_LOCK = drill 1.016 pad 1.88 octagon: 1 -1.397,5.08; 2 1.397,5.08; 3 -1.397,2.54; 4 1.397,2.54; 5 -1.397,0; 6 1.397,0; 7 -1.397,-2.54; 8 1.397,-2.54; 9 -1.397,-5.08; 10 1.397,-5.08
0805 = smd 1.2 x 1: 1 -1.1,0; 2 1.1,0
POWER-CHOKE_WE-TPC = smd 6.3 x 2.2: 1 0,2.05; 2 0,-2.05
CHIP-LED0805 = smd 1.2 x 1.2: A 0,-1.05; C 0,1.05
CARCASA_MOTOR_L_LOTTIE_LEMON = hole 3.2: 21.001,6.115; 11.443,45.812; 11.443,35.804; 15.059,6.115
B2B-PH_KL = drill 1.1 pad 1.5 long: 1 -1,0; 2 1,0
R0805 = smd 1.3 x 1.5: 1 -0.85,0; 2 0.85,0
SOT23 = smd 1 x 1.4: 1 -0.95,-1.1; 2 0.95,-1.1; 3 0,1.1
R0603-ROUND = smd 0.898 x 1.1: 1 -0.889,0; 2 0.889,0
CT/CN0603 = smd 1 x 1: 1 -1,0; 2 1,0
R1206 = smd 1.6 x 1.803: 1 -1.422,0; 2 1.422,0
CA9V = drill 1.321 long: A -2.54,-5.08; E 2.54,-5.08; S 0,5.08
TS42 = smd 1.6 x 1.4: 1 -4.2,2.25; 2 4.2,2.25; 3 -4.2,-2.25; 4 4.2,-2.25; 5 -4.2,0
CAY16 = smd 0.5 x 0.65: 1 -1.2,-0.675; 2 -0.4,-0.675; 3 0.4,-0.675; 4 1.2,-0.675; 5 1.2,0.675; 6 0.4,0.675; 7 -0.4,0.675; 8 -1.2,0.675
CARCASA_MOTOR_R_LOTTIE_LEMON = hole 3.2: -21.001,6.115; -11.443,45.712; -10.243,35.704; -15.059,6.115
GPI-152-3013 = drill 1.65: 10 -4.6,3.455; 11 -4.6,-3.455; 20 4.6,3.455; 21 4.6,-3.455; C@1 0,3.455; C@2 0,-3.455; P$7 11.43,4.85; P$8 -11.43,4.85; P$9 -11.43,-4.85; P$10 11.43,-4.85
SJL = smd 0.508 x 1.016: 1 -0.508,0; 2 0.508,0
SOT-23 = smd 0.787 x 0.889: 1 0.025,-1.016; 2 -0.94,1.016; 3 0.991,1.016
DPAK = smd 1.6 x 3: 1 -2.28,-4.04; 3 2.28,-4.04 | smd 4.826 x 4.191: 4 0,2.096
10X03MTA = drill 1.016 long: 1 2.54,0; 2 0,0; 3 -2.54,0
10X04MTA = drill 1.016 long: 1 3.81,0; 2 1.27,0; 3 -1.27,0; 4 -3.81,0
QFN44ML7X7 = smd 0.75 x 0.3: 1 -3.275,2.5; 2 -3.275,2; 3 -3.275,1.5; 4 -3.275,1; 5 -3.275,0.5; 6 -3.275,0; 7 -3.275,-0.5; 8 -3.275,-1; 9 -3.275,-1.5; 10 -3.275,-2; 11 -3.275,-2.5; 23 3.275,-2.5; 24 3.275,-2; 25 3.275,-1.5; 26 3.275,-1; 27 3.275,-0.5; 28 3.275,0; 29 3.275,0.5; 30 3.275,1; 31 3.275,1.5; 32 3.275,2; 33 3.275,2.5 | smd 0.3 x 0.75: 12 -2.5,-3.275; 13 -2,-3.275; 14 -1.5,-3.275; 15 -1,-3.275; 16 -0.5,-3.275; 17 0,-3.275; 18 0.5,-3.275; 19 1,-3.275; 20 1.5,-3.275; 21 2,-3.275; 22 2.5,-3.275; 34 2.5,3.275; 35 2,3.275; 36 1.5,3.275; 37 1,3.275; 38 0.5,3.275; 39 0,3.275; 40 -0.5,3.275; 41 -1,3.275; 42 -1.5,3.275; 43 -2,3.275; 44 -2.5,3.275 | smd 4.826 x 4.826: EXP 0,0
TQFP44-PAD = smd 1.4 x 0.45: 1 -5.8,4; 2 -5.8,3.2; 3 -5.8,2.4; 4 -5.8,1.6; 5 -5.8,0.8; 6 -5.8,0; 7 -5.8,-0.8; 8 -5.8,-1.6; 9 -5.8,-2.4; 10 -5.8,-3.2; 11 -5.8,-4; 23 5.8,-4; 24 5.8,-3.2; 25 5.8,-2.4; 26 5.8,-1.6; 27 5.8,-0.8; 28 5.8,0; 29 5.8,0.8; 30 5.8,1.6; 31 5.8,2.4; 32 5.8,3.2; 33 5.8,4 | smd 0.45 x 1.4: 12 -4,-5.8; 13 -3.2,-5.8; 14 -2.4,-5.8; 15 -1.6,-5.8; 16 -0.8,-5.8; 17 0,-5.8; 18 0.8,-5.8; 19 1.6,-5.8; 20 2.4,-5.8; 21 3.2,-5.8; 22 4,-5.8; 34 4,5.8; 35 3.2,5.8; 36 2.4,5.8; 37 1.6,5.8; 38 0.8,5.8; 39 0,5.8; 40 -0.8,5.8; 41 -1.6,5.8; 42 -2.4,5.8; 43 -3.2,5.8; 44 -4,5.8 | smd 1 x 1: P$1 0,0
BASE_ROBOT_001 = hole 3.2: 5.08,91.44; 152.4,152.4; 30.48,152.4; 177.8,91.44; 30.48,30.48; 152.4,30.48; 58.42,171.196; 124.46,171.196; 58.42,11.659; 124.46,11.659; 25.375,139.7; 25.375,43.18; 157.455,139.7; 157.455,43.18
PADS_LOTTIE_LEMON = drill 1 pad 1.93: P$1 0,0; P$2 2.54,0; P$3 0,2.54; P$4 2.54,2.54; P$5 2.54,5.08; P$6 5.08,5.08; P$7 5.08,2.54; P$8 5.08,0; P$9 7.62,0; P$10 7.62,2.54; P$11 10.16,5.08; P$12 10.16,2.54; P$13 10.16,0; P$14 5.08,10.16; P$15 10.16,10.16; P$16 7.62,12.7; P$17 10.16,12.7; P$18 12.7,15.24; P$19 12.7,12.7; P$20 12.7,10.16; P$21 12.7,7.62; P$22 12.7,5.08; P$23 12.7,2.54; P$24 12.7,0; P$25 15.24,15.24; P$26 15.24,12.7; P$27 15.24,10.16; P$28 15.24,7.62; P$29 15.24,5.08; P$30 15.24,2.54; P$31 15.24,0; P$32 17.78,22.86; P$33 17.78,20.32; P$34 17.78,17.78; P$35 17.78,15.24; P$36 17.78,12.7; P$37 17.78,10.16; P$38 17.78,7.62; P$39 17.78,5.08; P$40 17.78,2.54; P$41 17.78,0; P$42 20.32,25.4; P$43 20.32,22.86; P$44 22.86,20.32; P$45 20.32,20.32; P$46 20.32,17.78; P$47 20.32,15.24; P$48 20.32,12.7; P$49 20.32,10.16; P$50 20.32,5.08; P$51 20.32,7.62; P$52 20.32,0; P$53 20.32,2.54; P$54 22.86,27.94; P$55 22.86,25.4; P$56 22.86,22.86; P$57 22.86,17.78; P$58 22.86,15.24; P$59 22.86,12.7; P$60 22.86,10.16; P$61 22.86,7.62; P$62 22.86,5.08; P$63 22.86,2.54; P$64 22.86,0; P$65 25.4,30.48; P$66 25.4,27.94; P$67 25.4,25.4; P$68 25.4,22.86; P$69 25.4,20.32; P$70 25.4,17.78; P$71 25.4,15.24; P$72 25.4,12.7; P$73 25.4,10.16; P$74 25.4,7.62; P$75 25.4,5.08; P$76 25.4,2.54; P$77 25.4,0; P$78 27.94,30.48; P$79 27.94,27.94; P$80 27.94,25.4; P$81 27.94,22.86; P$82 27.94,20.32; P$83 27.94,17.78; P$84 27.94,15.24; P$85 27.94,12.7; P$86 27.94,10.16; P$87 27.94,7.62; P$88 27.94,5.08; P$89 27.94,2.54; P$90 27.94,0; P$91 109.22,30.48; P$92 30.48,30.48; P$93 30.48,27.94; P$94 30.48,25.4; P$95 30.48,22.86; P$96 30.48,17.78; P$97 30.48,20.32; P$98 30.48,12.7; P$99 30.48,15.24; P$100 30.48,10.16; P$101 30.48,7.62; P$102 30.48,5.08; P$103 30.48,2.54; P$104 30.48,0; P$105 106.68,30.48; P$106 33.02,30.48; P$107 33.02,27.94; P$108 33.02,25.4; P$109 33.02,22.86; P$110 33.02,20.32; P$111 33.02,17.78; P$112 106.68,27.94; P$113 35.56,30.48; P$114 35.56,27.94; P$115 35.56,25.4; P$116 35.56,22.86; P$117 35.56,20.32; P$118 38.1,20.32; P$119 38.1,22.86; P$120 38.1,25.4; P$121 38.1,27.94; P$122 38.1,30.48; P$123 106.68,25.4; P$124 40.64,20.32; P$125 40.64,22.86; P$126 40.64,25.4; P$127 40.64,27.94; P$128 40.64,30.48; P$129 106.68,22.86; P$130 43.18,20.32; P$131 43.18,22.86; P$132 43.18,25.4; P$133 43.18,27.94; P$134 43.18,30.48; P$135 104.14,25.4; P$136 45.72,20.32; P$137 45.72,22.86; P$138 45.72,25.4; P$139 45.72,27.94; P$140 45.72,30.48; P$141 104.14,27.94; P$142 48.26,20.32; P$143 48.26,22.86; P$144 48.26,25.4; P$145 48.26,27.94; P$146 48.26,30.48; P$147 101.6,30.48; P$148 50.8,30.48; P$149 50.8,27.94; P$150 50.8,25.4; P$151 50.8,22.86; P$152 104.14,30.48; P$153 53.34,30.48; P$154 53.34,27.94; P$155 53.34,25.4; P$156 101.6,27.94; P$157 101.6,25.4; P$158 104.14,22.86; P$159 109.22,20.32; P$160 106.68,20.32; P$161 99.06,30.48; P$162 99.06,27.94; P$163 99.06,25.4; P$164 96.52,25.4; P$165 96.52,27.94; P$166 93.98,30.48; P$167 96.52,30.48; P$168 93.98,27.94; P$169 93.98,25.4; P$170 101.6,22.86; P$171 99.06,22.86; P$172 96.52,22.86; P$173 99.06,20.32; P$174 111.76,20.32; P$175 101.6,20.32; P$176 104.14,20.32; P$177 114.3,15.24; P$178 111.76,17.78; P$179 111.76,22.86; P$180 111.76,25.4; P$181 109.22,17.78; P$182 111.76,15.24; P$183 114.3,12.7; P$184 33.02,15.24; P$185 35.56,17.78; P$186 38.1,17.78; P$187 35.56,15.24; P$188 33.02,12.7; P$189 111.76,27.94; P$190 111.76,30.48; P$199 109.22,25.4; P$200 109.22,22.86; P$201 114.3,30.48; P$202 114.3,27.94; P$203 114.3,25.4; P$204 114.3,22.86; P$205 114.3,20.32; P$206 114.3,17.78; P$207 109.22,27.94; P$208 116.84,30.48; P$209 116.84,27.94; P$210 116.84,25.4; P$211 116.84,22.86; P$212 116.84,20.32; P$213 116.84,17.78; P$214 116.84,15.24; P$215 116.84,12.7; P$216 116.84,10.16; P$217 116.84,7.62; P$218 116.84,5.08; P$219 116.84,2.54; P$220 116.84,0; P$221 119.38,30.48; P$222 119.38,27.94; P$223 119.38,25.4; P$224 119.38,22.86; P$225 119.38,20.32; P$226 119.38,17.78; P$227 119.38,15.24; P$228 119.38,12.7; P$229 119.38,10.16; P$230 119.38,7.62; P$231 119.38,5.08; P$232 119.38,2.54; P$233 119.38,0; P$234 121.92,30.48; P$235 121.92,27.94; P$236 121.92,25.4; P$237 121.92,22.86; P$238 121.92,20.32; P$239 121.92,17.78; P$240 121.92,15.24; P$241 121.92,12.7; P$242 121.92,10.16; P$243 121.92,7.62; P$244 121.92,5.08; P$245 121.92,2.54; P$246 121.92,0; P$247 124.46,27.94; P$248 124.46,25.4; P$249 124.46,22.86; P$250 124.46,20.32; P$251 124.46,15.24; P$252 124.46,17.78; P$253 124.46,12.7; P$254 124.46,10.16; P$255 124.46,7.62; P$256 124.46,5.08; P$257 124.46,2.54; P$258 124.46,0; P$259 127,25.4; P$260 127,22.86; P$261 127,20.32; P$262 127,17.78; P$263 127,15.24; P$264 127,12.7; P$265 127,10.16; P$266 127,7.62; P$267 127,5.08; P$268 127,2.54; P$269 127,0; P$270 129.54,22.86; P$271 129.54,20.32; P$272 129.54,17.78; P$273 129.54,15.24; P$274 129.54,12.7; P$275 129.54,10.16; P$276 129.54,7.62; P$277 129.54,5.08; P$278 129.54,2.54; P$279 129.54,0; P$280 132.08,15.24; P$281 132.08,12.7; P$282 132.08,10.16; P$283 132.08,7.62; P$284 132.08,5.08; P$285 132.08,2.54; P$286 132.08,0; P$287 134.62,15.24; P$288 134.62,12.7; P$289 134.62,10.16; P$290 134.62,7.62; P$291 134.62,5.08; P$292 134.62,2.54; P$293 134.62,0; P$294 137.16,12.7; P$295 137.16,10.16; P$296 137.16,5.08; P$297 137.16,2.54; P$298 137.16,0; P$299 139.7,12.7; P$300 139.7,2.54; P$301 139.7,0; P$302 142.24,10.16; P$303 142.24,5.08; P$304 142.24,2.54; P$305 142.24,0; P$306 144.78,5.08; P$307 144.78,2.54; P$308 144.78,0; P$309 147.32,2.54; P$310 147.32,0
CRYSTAL-3.2-2.5 = smd 1.3 x 1.05: 1 -1.15,-0.925; 2 1.15,-0.925; 3 1.15,0.925; 4 -1.15,0.925
PN61729 = drill 0.95 pad 1.676 octagon: 1 1.25,4.71; 2 -1.25,4.71; 3 -1.25,2.71; 4 1.25,2.71 | drill 2.2: P$1 -6,0; P$2 6,0

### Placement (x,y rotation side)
B2  113.61,33.02 180 top
BB1  91.44,7.62 0 top
BB2  91.44,161.3 0 top
C1  79.25,43.94 270 top
C2  87.38,31.75 90 top
C3  57.1,135.33 270 top
C4  94.74,31.75 270 top
C5  88.65,53.09 180 top
C6  97.54,51.82 90 top
C7  71.93,141.63 270 top
C8  74.93,43.94 270 top
C9  81.53,43.94 90 top
C10  85.95,143.05 270 top
C11  140.82,69.7 180 top
C12  101.19,142.04 270 top
C13  172.72,21.59 180 top
C14  137.36,52.83 180 top
C15  117.65,135.94 270 top
C16  100.84,73.15 270 top
C17  82.04,73.15 90 top
C18  12.14,161.95 90 top
C19  10.46,170.08 90 top
C20  74.32,114.15 90 top
C21  5.74,161.34 90 top
C22  65.58,121.51 90 top
C23  66.4,115.32 90 top
C24  20.42,164.64 90 top
C25  60.96,37.34 90 top
C26  60.96,30.73 270 top
C27  76.96,77.22 270 top
C28  56.08,121.31 180 top
C29  not placed on the board
C30  not placed on the board
C31  not placed on the board
C32  not placed on the board
C33  not placed on the board
C34  34.04,115.32 0 top
C35  43.69,107.7 180 top
C36  34.04,107.7 0 top
C37  168.66,12.19 270 top
C38  175.51,11.94 270 top
C39  138.33,17.53 90 top
C40  130.86,29.92 90 top
C41  not placed on the board
C42  not placed on the board
C44  not placed on the board
C45  not placed on the board
CHRG  135.64,16.51 90 top
CM1  53.59,77.47 90 top
CM2  53.59,74.17 90 top
D1  69.09,35.05 90 top
D2  157.89,7.92 90 top
D3  132.38,24.43 180 bottom
D4  75.64,107.29 90 top
DZ1  not placed on the board
F1  56.64,34.04 90 top
FM1  124.56,166.17 0 top
FM2  144.32,97.28 0 top
FM3  78.69,173.94 0 top
FR1  51.56,47.8 270 top
FS1  63.2,137.16 0 top
FS2  77.42,142.85 0 top
FS3  91.44,143.52 0 top
FS4  106.67,143.52 0 top
FS5  123.3,137.35 0 top
HB  91.44,111.21 270 top
IC1  129.29,122.94 90 top
IC2  64,75.64 270 top
IC3  129.29,112.27 90 top
IC4  91.44,67.56 90 top
IC5  56.49,126.75 0 top
IC6  70.41,117.6 0 top
IC7  125.88,63.86 270 top
IC8  73.16,60.16 270 top
IC9  68.33,110.03 90 top
J1  66.04,10.92 0 top
JP1  113.43,15 180 top
JP2  118.97,42.11 90 top
L1  76.96,43.94 90 top
L2  44.96,34.04 270 top
L3  46.33,126.24 90 top
L4  136.14,26.67 270 top
LED1  63.2,142.65 90 top
LED2  77.42,148.34 90 top
LED3  91.44,149.35 90 top
LED4  105.87,149.56 270 top
LED5  123.34,143.05 90 top
LL1  153.96,102.46 180 top
MA  129.91,80.29 0 top
MB  55.27,65.58 0 top
NM  not placed on the board
NM1  128.27,47.5 0 top
NM2  127.91,74.21 0 top
NM3  78.99,49.78 0 top
NM4  88.14,55.37 0 top
NM5  4.47,167.84 0 top
ON  133.1,16.51 90 top
Q1  41.96,175.92 180 top
R1  66.04,34.8 270 top
R2  54.25,135.33 270 top
R3  57.1,138.99 270 top
R4  91.03,35.05 0 top
R5  54.25,138.99 90 top
R6  99.57,51.82 270 top
R7  69.29,141.63 270 top
R8  71.93,145.08 90 top
R9  69.29,145.08 90 top
R10  53.09,34.04 90 top
R11  46.99,34.04 90 top
R12  55.88,131.67 0 top
R13  83.31,143.05 270 top
R14  86.16,147.12 90 top
R15  83.31,147.12 90 top
R16  153.31,41.86 180 top
R17  98.55,142.04 270 top
R18  101.19,145.49 270 top
R19  98.55,145.69 90 top
R20  83.57,69.6 0 top
R21  100.08,67.06 90 top
R22  114.6,135.94 270 top
R23  117.65,139.6 270 top
R24  114.6,139.6 90 top
R25  98.3,73.15 90 top
R26  84.58,73.15 270 top
R27  95.76,73.15 270 top
R28  87.12,73.15 90 top
R29  63.5,109.37 0 top
R30  93.22,73.15 90 top
R31  89.66,73.15 270 top
R32  70.1,114.45 180 top
R33  16.36,165.25 90 top
R34  51.82,123.75 90 top
R35  51.82,131.47 0 top
R36  29.87,166.07 90 top
R37  22.25,168.76 90 top
R38  25.2,172.36 0 top
R39  130.3,17.53 90 top
R40  128.02,17.53 270 top
R41  80.06,28.91 0 top
R42  65.53,58.67 90 top
R43  65.53,55.37 90 top
R44  143.27,30.47 180 top
R45  51,128.83 90 top
R46  10.26,156.11 90 top
RESET  74.17,35.05 90 top
RN1  50.04,34.04 0 top
RN2  124.56,58.32 0 top
RN3  not placed on the board
RR1  29.46,102.46 180 top
S1  91.44,21.6 180 top
SJ1  not placed on the board
SJ2  not placed on the board
T1  140.61,53.85 270 top
T2  159,36.37 90 top
T3  79.96,31.9 270 top
T4  132.84,24.64 0 top
T5  61.98,47.75 90 top
TK1  5.08,83.92 270 top
TK2  52.02,168.66 180 top
TK3  131.67,168.45 180 top
TK4  177.8,83.92 90 top
TWI  147.27,45.92 0 top
U1  91.44,43.43 0 top
U2  91.44,43.43 0 top
U$1  0,0 0 top
U$2  17.78,132.08 0 top
W1  154.93,55.89 0 top
W2  10.16,55.89 0 top
X1  91.03,31.75 180 top
X2  48.39,23.12 327.5 top

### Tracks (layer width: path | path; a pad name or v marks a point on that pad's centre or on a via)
+3V3  (4 unrouted)
+5V  (via drill 0.41)  (37 unrouted)
  Top 0.254: U1.34 93.94,46.95 95.44,48.45 U2.34 | U1.2 87.66,45.43 86.46,46.63 U2.2 | U1.14 89.94,39.39 89.04,38.49 U2.14
  Top 0.305: U2.2 80.16,46.63 79.25,45.72 C1.1
  Top 0.406: R1.2 67.18,33.91 67.74,33.35 D1.C | U2.34 95.44,51.75 96.39,52.7 C6.2 | S1.10 96.04,16.28 94.49,14.73 80.52,14.73
  Bottom 0.305: J1.2 66.04,14.48 66.8,15.24 v67.06,33.78
+BAT_M  (8 unrouted)
+VB  (10 unrouted)
  Top 0.406: S1.11 96.04,23.4 94.49,21.84 59.69,21.84 54.1,16.26 46.74,16.26 39.12,23.88 39.12,44.45
  Top 1.27: C35.+ C36.+ C34.+
+VBC  (3 unrouted)
+VDC  (1 unrouted)
+VDCI  (12 unrouted)
AD0/TK1  (2 unrouted)
  Top 0.305: U2.36 93.84,50.15 94.23,50.55
AD1/TK2  (via drill 0.41)  (1 unrouted)
  Top 0.254: U1.37 92.44,47.74 93.04,48.34 U2.37
  Top 0.305: U2.37 93.04,50.11 93.47,50.55 93.47,52.32 v92.96,52.83
  Bottom 0.305: v92.96,52.83 92.96,109.98
AD2/MUX  (via drill 0.41)  (1 unrouted)
  Top 0.254: U1.38 91.94,48 92.24,48.3 U2.38
  Top 0.305: U2.38 92.24,50.33 92.71,50.8 92.71,51.56 v92.2,52.07
  Bottom 0.305: v92.2,52.07 92.2,110.24
AD3/TRIM  (via drill 0.41)  (1 unrouted)
  Top 0.305: v91.95,51.05 91.44,50.55 U2.39 U1.39
  Bottom 0.305: v91.95,51.05 91.44,50.55 91.44,33.53
AD4/CSA  (1 unrouted)
  Top 0.254: U1.40 90.94,48 90.64,48.3 U2.40
  Top 0.305: U2.40 90.64,51.02 91.44,51.82 91.44,64.77 | IC4.1 95.27,65.56 95.76,66.04 R27.2 R25.1 C16.2
AD5/CSB  (2 unrouted)
  Top 0.254: U1.41 90.44,47.74 89.84,48.34 U2.41
  Top 0.305: U2.41 89.84,51.23 90.68,52.07 90.68,66.29 | R28.2 R26.1 C17.2
AGND  (2 unrouted)
  Top 0.254: U1.43 89.44,47.21 88.24,48.41 U2.43
AN0  (4 unrouted)
AN1  (4 unrouted)
AN2  (4 unrouted)
AN3  (4 unrouted)
AN4  (4 unrouted)
AREF  (1 unrouted)
  Top 0.254: U1.42 89.94,47.47 89.04,48.37 U2.42
AVC  (3 unrouted)
  Top 0.254: U1.24 95.22,41.43 96.42,40.23 U2.24 | U1.44 88.93,46.71 87.44,48.2 U2.44
  Top 0.305: 87.44,48.2 87.38,48.26
CHRG  (2 unrouted)
D+  (via drill 0.41)
  Top 0.254: U1.4 87.14,44.43 86.54,45.03 U2.4
  Top 0.305: U2.4 83.64,45.03 v83.57,44.96 | RN1.8 48.84,35.63 v49.02,35.81
  Bottom 0.305: v83.57,44.96 73.15,44.96 68.83,40.64 52.07,40.64 49.02,37.59 v49.02,35.81
D-  (via drill 0.41)
  Top 0.254: U1.3 87.4,44.93 86.5,45.83 U2.3
  Top 0.305: U2.3 83.71,45.83 v83.57,45.97 | v68.07,41.4 54.1,41.4 v51.05,38.35 | RN1.5 51.24,35.63 v51.05,35.81
  Bottom 0.305: v83.57,45.97 72.64,45.97 v68.07,41.4 | v51.05,38.35 v51.05,35.81
DIO4/TK3  (via drill 0.41)  (1 unrouted)
  Top 0.254: U1.25 95.48,41.93 96.38,41.03 U2.25
  Top 0.305: U2.25 98.16,41.03 v98.81,40.39
  Bottom 0.305: v98.81,40.39 98.04,41.15 98.04,47.24 102.87,52.07 102.87,157.73 109.98,164.85
DIO5/INA2  (via drill 0.41)  (1 unrouted)
  Top 0.254: U1.31 95.48,44.93 96.38,45.83 U2.31
  Top 0.305: U2.31 102.25,45.83 v102.62,45.47
  Bottom 0.305: v102.62,45.47 103.12,45.47 107.44,49.78 112.01,49.78 115.32,53.09
DIO6/INA1  (via drill 0.41)  (1 unrouted)
  Top 0.254: U1.27 96,42.93 96.3,42.63 U2.27
  Top 0.305: U2.27 99.35,42.63 v99.82,42.16
  Bottom 0.305: v99.82,42.16 103.89,42.16 108.46,46.74 113.03,46.74 118.36,52.07 118.36,74.42
DIO7/MUXA  (via drill 0.41)  (1 unrouted)
  Top 0.254: U1.1 87.92,45.93 86.42,47.43 U2.1
  Top 0.305: 86.42,47.43 84.39,47.43 v84.07,47.75
  Bottom 0.305: v84.07,47.75 97.54,47.75 102.11,52.32 102.11,113.79
DIO8/MUXB  (via drill 0.41)  (1 unrouted)
  Top 0.254: U1.28 U2.28
  Top 0.305: U2.28 100.08,43.43 v100.58,42.93
  Bottom 0.305: v100.58,42.93 103.63,42.93 108.2,47.5 112.78,47.5 117.6,52.32 117.6,117.35 121.16,120.9
DIO9/INB2  (via drill 0.41)  (1 unrouted)
  Top 0.254: U1.29 96,43.93 96.3,44.23 U2.29
  Top 0.305: U2.29 100.8,44.23 v101.35,43.69
  Bottom 0.305: v101.35,43.69 103.38,43.69 107.95,48.26 112.52,48.26 116.84,52.58 116.84,69.6 115.57,70.87
DIO10/INB1  (via drill 0.41)  (1 unrouted)
  Top 0.254: U1.30 95.74,44.43 96.34,45.03 U2.30
  Top 0.305: U2.30 101.52,45.03 v102.11,44.45
  Bottom 0.305: v102.11,44.45 103.12,44.45 107.7,49.02 112.27,49.02 116.08,52.83 116.08,69.09 115.32,69.85
DIO11/MUXC  (1 unrouted)
  Top 0.254: U1.12 88.94,39.92 87.44,38.42 U2.12
DIO12/TK4  (via drill 0.41)  (1 unrouted)
  Top 0.254: U1.26 95.74,42.43 96.34,41.83 U2.26
  Top 0.305: U2.26 98.63,41.83 v99.06,41.4
  Bottom 0.305: v99.06,41.4 104.14,41.4 108.71,45.97 137.41,45.97 140.72,49.28 167.39,49.28 174.24,56.13
DIO13/MUXI  (via drill 0.41)  (1 unrouted)
  Top 0.254: U1.32 95.22,45.43 96.42,46.63 U2.32
  Top 0.305: U2.32 102.77,46.63 v103.12,46.99
  Bottom 0.305: v103.12,46.99 103.63,46.99 107.19,50.55 111.76,50.55 114.55,53.34 114.55,67.82 112.27,70.1 112.27,114.05 119.38,121.16
EN  (3 unrouted)
GND  (111 unrouted)
  Top 0.254: U1.15 90.44,39.13 89.84,38.53 U2.15 | U1.35 93.44,47.21 94.64,48.41 U2.35
  Top 0.279: U1.23 94.72,40.41 94.74,40.39 95.25,40.39 96.2,39.43 U2.23
  Top 0.305: RESET.3 76.42,33.75 76.96,34.29 76.96,36.07 76.42,36.61 RESET.4
GNDA  (3 unrouted)
HWB
  Top 0.254: U1.33 94.96,45.93 96.46,47.43 U2.33
  Top 0.406: U2.33 98.49,47.43 99.57,48.51 R6.2
MISO  (via drill 0.41)  (1 unrouted)
  Top 0.254: U1.11 87.92,40.93 86.42,39.43 U2.11
  Top 0.305: U2.11 83.25,39.43 v82.8,39.88
  Bottom 0.305: v82.8,39.88 74.42,39.88 72.9,38.35 72.9,33.78 71.63,32.51
MOSI  (via drill 0.41)  (1 unrouted)
  Top 0.254: U1.10 87.66,41.43 86.46,40.23 U2.10
  Top 0.305: U2.10 83.97,40.23 v83.57,40.64
  Bottom 0.305: v83.57,40.64 74.42,40.64 72.39,38.61
N$1  (1 unrouted)
N$3  (1 unrouted)
N$4
  Bottom 1.27: B2.AC2 116.15,26.24 113.54,23.62 113.54,21.38 JP1.2
N$5  (1 unrouted)
N$6  (1 unrouted)
N$7
  Bottom 1.27: B2.AC1 111.07,28.52 108.46,25.91 108.46,17.27 110.38,15.35 JP1.3 116.5,18.35 JP1.1
N$9
  Top 0.406: R11.2 45.06,35.04 L2.1
  Top 0.508: R11.2 46.99,36.32 47.75,37.08 52.32,37.08 53.09,36.32 R10.2
  Top 0.61: L2.1 44.03,35.14 43.18,34.29 43.18,26.49 X2.P$1 43.33,24.49 47.92,19.9 X2.P$2
N$11  (2 unrouted)
N$12  (1 unrouted)
N$13  (2 unrouted)
N$14  (1 unrouted)
N$15  (1 unrouted)
N$16  (1 unrouted)
N$17  (1 unrouted)
N$18  (1 unrouted)
N$19  (1 unrouted)
N$20  (1 unrouted)
N$21  (2 unrouted)
N$22  (1 unrouted)
N$23  (1 unrouted)
N$24  (1 unrouted)
N$25  (1 unrouted)
N$26  (1 unrouted)
N$27  (1 unrouted)
N$28  (1 unrouted)
  Top 0.305: 90.93,68.58 90.93,71.88 90.55,72.26 R31.2 88.77,72.26 87.88,73.15 85.47,73.15 R26.2 C17.1
N$29  (1 unrouted)
  Top 0.305: 91.95,67.31 91.95,73.41 92.58,74.04 R30.2 93.85,74.04 94.74,73.15 97.41,73.15 R25.2 C16.1
N$30  (1 unrouted)
N$31  (1 unrouted)
N$32  (1 unrouted)
N$33  (4 unrouted)
N$34  (2 unrouted)
N$35  (1 unrouted)
N$36  (1 unrouted)
N$37  (1 unrouted)
N$38  (1 unrouted)
N$39  (3 unrouted)
N$40  (1 unrouted)
N$41  (1 unrouted)
N$42  (1 unrouted)
N$43  (1 unrouted)
N$44  (2 unrouted)
N$45  (2 unrouted)
N$46  (1 unrouted)
N$47  (1 unrouted)
N$48  (2 unrouted)
N$49  (1 unrouted)
N$50  (2 unrouted)
N$51
  Top 0.356: RN1.1 48.84,32 | 48.84,32 48.84,31.43 49.28,30.99 | R11.1 47.81,33.04 48.84,32
  Top 0.508: X2.3 47.75,27.12 47.75,27.94 49.28,29.46 49.28,30.99
N$52  (2 unrouted)
N$53  (1 unrouted)
N$54
  Top 0.356: RN1.4 51.24,32 | 51.24,32 51.24,31.43 50.8,30.99 | R10.1 52.27,33.04 51.24,32
  Top 0.508: X2.2 50.8,28.7 50.8,30.99
N$55  (1 unrouted)
N$56  (1 unrouted)
ON  (2 unrouted)
OUT1  (3 unrouted)
OUT2  (3 unrouted)
OUT3  (3 unrouted)
OUT4  (3 unrouted)
RESET  (via drill 0.41)
  Top 0.254: U1.13 89.44,39.66 88.24,38.46 U2.13
  Top 0.305: RESET.1 71.92,29.25 v71.88,29.21 | U2.13 88.24,36.42 v87.88,36.07
  Top 0.406: R1.1 68.02,35.69 D1.A | RESET.1 71.92,33.49 71.37,34.04 71.37,36.07 71.92,36.61 RESET.2
  Top 0.61: D1.A 69.09,38.35 69.99,39.25 RESET.2
  Bottom 0.305: J1.5 72.64,12.45 72.64,14.22 71.88,14.99 v71.88,29.21 71.92,29.25 71.92,32 75.98,36.07 v87.88,36.07
RX  (via drill 0.41)  (1 unrouted)
  Top 0.254: U1.20 92.94,39.39 93.84,38.49 U2.20
  Top 0.305: 93.84,38.49 93.84,35.95 v95.5,34.29
  Bottom 0.305: v95.5,34.29 102.11,34.29 109.04,41.48
SCK  (via drill 0.41)  (1 unrouted)
  Top 0.254: U1.9 87.4,41.93 86.5,41.03 U2.9
  Top 0.305: U2.9 84.7,41.03 v84.33,41.4
  Bottom 0.305: v84.33,41.4 74.42,41.4 72.14,39.12
SCL  (via drill 0.41)  (1 unrouted)
  Top 0.305: U2.18 92.24,36.03 v92.96,35.31
  Bottom 0.305: v92.96,35.31 94.23,35.31 95.25,35.81 101.6,35.81 110.49,44.96 138.68,44.96 141.73,48.01 143,48.01 143.46,47.55 TWI.4
SDA  (via drill 0.41)  (1 unrouted)
  Top 0.305: U1.19 92.44,40.88 93.22,41.66 | U2.19 v93.04,36.3 | v93.04,36.3
  Bottom 0.305: v93.04,36.3 94.46,36.3 95,36.83 101.85,36.83 108.71,43.69 108.97,43.69 110.74,45.47 137.92,45.47 140.97,48.51 145.29,48.51 146,47.8 TWI.3
SENA  (2 unrouted)
SENB  (2 unrouted)
SS/RXLED
  Top 0.254: U1.8 87.14,42.43 86.54,41.83 U2.8
TX  (via drill 0.41)
  Top 0.254: U1.21 93.44,39.66 94.64,38.46 U2.21
  Top 0.305: 94.64,38.46 94.64,36.68 v96.27,35.05
  Bottom 0.305: v96.27,35.05 101.85,35.05 110.74,44.2 115.06,44.7 116.43,44.35 JP2.4
TXLED
  Top 0.254: U1.22 93.94,39.92 95.44,38.42 U2.22
UCAP
  Top 0.254: U1.6 U2.6
  Top 0.305: U2.6 81.91,43.43 C9.1
UGND  (2 unrouted)
  Top 0.254: U1.5 86.88,43.93 86.58,44.23 U2.5
  Top 0.305: U2.5 82.13,44.23 C9.2
  Top 0.406: X2.4 50.29,24.13 47.75,24.13 46.74,25.15 46.74,30.23 44.96,32 L2.2
VIN  (2 unrouted)
VINA  (4 unrouted)
VUSB  (via drill 0.41)  (9 unrouted)
  Top 0.254: U1.7 86.88,42.93 86.58,42.63 U2.7
  Top 0.305: U2.7 84.04,42.63 v83.57,42.16 | v60.96,37.34 C25.+
  Top 0.762: F1.2 60.81,35.99 C25.+ C26.+
  Bottom 0.305: v83.57,42.16 74.42,42.16 70.36,38.1 63.5,38.1 62.74,37.34 v60.96,37.34
X1
  Top 0.254: U1.17 U2.17
  Top 0.305: 92.22,32.64 X1.1 91.92,32.94
  Top 0.356: U2.17 91.44,35.53 R4.2 91.92,32.94 | C4.1 92.22,32.64
X2
  Top 0.254: U1.16 90.94,38.87 90.64,38.57 U2.16
  Top 0.305: R4.1 90.14,34.34 91.01,33.48 91.01,31.06 90.77,30.82 X1.3
  Top 0.356: U2.16 90.64,35.55 R4.1 | C2.1 89.85,30.86 X1.3
XUSB
  Top 0.762: X2.1 51.97,29.62 54.44,32.09 F1.1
